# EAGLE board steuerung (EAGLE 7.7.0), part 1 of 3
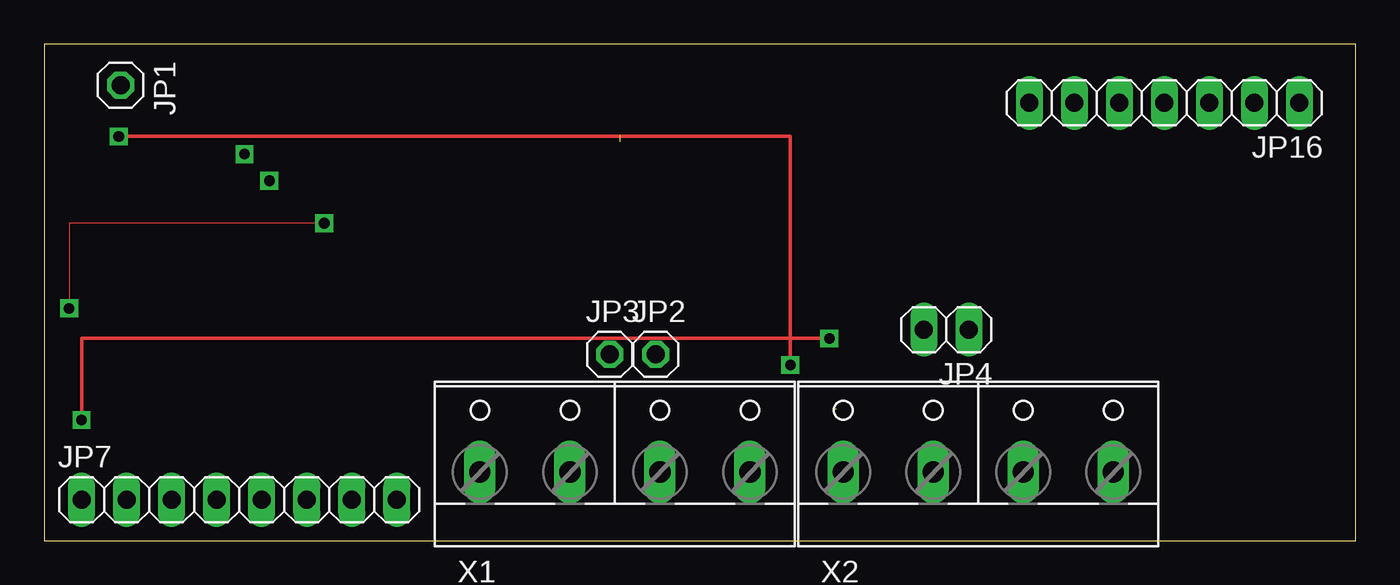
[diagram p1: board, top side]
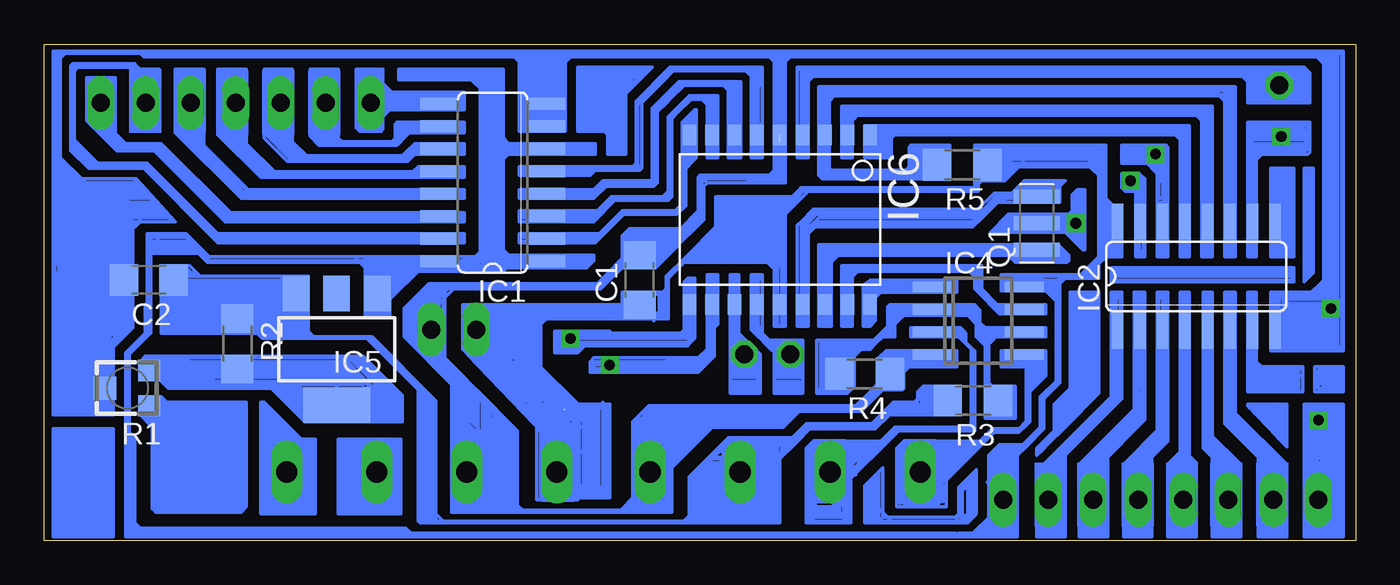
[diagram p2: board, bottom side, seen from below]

Size 74 x 28 mm. Coordinates in mm from the lower left corner, seen from the top.
Outline: 0,0 74,0 74,28 0,28 0,0
Copper layers (1*16): Top 0.035mm / dielectric 1.5mm / Bottom 0.035mm
Design rules "default": minimum track width 10mil, minimum drill 24mil, track to track 8mil, track to pad 8mil, pad to pad 8mil, via to via 8mil, smd to smd 8mil, copper to edge 40mil, drill to drill 8mil, minimum pad ring 10mil, minimum via ring 8mil, stop-mask expansion 4mil, vias tented up to drill 0mil, thermal gap 10mil

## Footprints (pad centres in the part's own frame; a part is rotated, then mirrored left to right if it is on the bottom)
C1206 = smd 1.6 x 1.8: 1 -1.4,0; 2 1.4,0
SO16 = smd 0.66 x 2.032: 1 -4.445,-3.073; 2 -3.175,-3.073; 3 -1.905,-3.073; 4 -0.635,-3.073; 5 0.635,-3.073; 6 1.905,-3.073; 7 3.175,-3.073; 8 4.445,-3.073; 9 4.445,3.073; 10 3.175,3.073; 11 1.905,3.073; 12 0.635,3.073; 13 -0.635,3.073; 14 -1.905,3.073; 15 -3.175,3.073; 16 -4.445,3.073
SO08 = smd 0.6 x 2.2: 1 -1.905,-2.6; 2 -0.635,-2.6; 3 0.635,-2.6; 4 1.905,-2.6; 5 1.905,2.6; 6 0.635,2.6; 7 -0.635,2.6; 8 -1.905,2.6
SOT223 = smd 1.5 x 2: 1 -2.3,-3.15; 2 0,-3.15; 3 2.3,-3.15 | smd 3.8 x 2: 4 0,3.15
SO-18W = smd 0.762 x 1.143: 1 -5.08,-4.788; 2 -3.81,-4.788; 3 -2.54,-4.788; 4 -1.27,-4.788; 5 0,-4.788; 6 1.27,-4.788; 7 2.54,-4.788; 8 3.81,-4.788; 9 5.08,-4.788; 10 5.08,4.788; 11 3.81,4.788; 12 2.54,4.788; 13 1.27,4.788; 14 0,4.788; 15 -1.27,4.788; 16 -2.54,4.788; 17 -3.81,4.788; 18 -5.08,4.788
1X01 = drill 1.016 octagon: 1 0,0
1X02 = drill 1.016 long: 1 -1.27,0; 2 1.27,0
1X08 = drill 1.016 long: 1 -8.89,0; 2 -6.35,0; 3 -3.81,0; 4 -1.27,0; 5 1.27,0; 6 3.81,0; 7 6.35,0; 8 8.89,0
1X07 = drill 1.016 long: 1 -7.62,0; 2 -5.08,0; 3 -2.54,0; 4 0,0; 5 2.54,0; 6 5.08,0; 7 7.62,0
CSTCR6M = smd 0.8 x 2.6: 1 -1.5,0; 2 0,0; 3 1.5,0
RTRIM3103 = smd 1.2 x 1.25: 1 -1,-1.225; 3 1,-1.225 | smd 1.3 x 1.3: 2 0,1.3
R1206 = smd 1.6 x 1.803: 1 -1.422,0; 2 1.422,0
W237-4P = drill 1.194 long: 1 -7.62,-0.635; 2 -2.54,-0.635; 3 2.54,-0.635; 4 7.62,-0.635

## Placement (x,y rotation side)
C1  100n  [C1206]  40.4,14.7 90 bottom
C2  100n  [C1206]  68.1,14.7 180 bottom
IC1  4543D  [SO16]  48.7,20.2 90 bottom
IC2  4028D  [SO16]  9,14.9 0 bottom
IC4  LM358D  [SO08]  21.3,12.4 270 bottom
IC5  LM317  [SOT223]  57.5,10.8 180 bottom
IC6  PIC18F1220SO  [SO-18W]  32.5,18.1 180 bottom
JP1  [1X01]  4.3,25.7 270 top
JP2  [1X01]  34.5,10.5 0 top
JP3  [1X01]  31.9,10.5 0 top
JP4  [1X02]  50.9,11.9 180 top
JP7  [1X08]  11,2.3 0 top
JP16  [1X07]  63.2,24.7 180 top
Q1  CSTCR6M00G53Z  [CSTCR6M]  18,17.9 90 bottom
R1  5k  [RTRIM3103]  69.3,8.6 90 bottom
R2  220  [R1206]  63.1,11.1 270 bottom
R3  10k  [R1206]  21.6,7.9 180 bottom
R4  10k  [R1206]  27.7,9.4 180 bottom
R5  1k  [R1206]  22.2,21.2 180 bottom
X1  [W237-4P]  32.2,4.5 0 top
X2  [W237-4P]  52.7,4.5 0 top

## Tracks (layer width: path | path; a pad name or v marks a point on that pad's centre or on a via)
N$1
  Bottom 0.2: 70.5,25.8 70.1,25.8 | 70.1,25.8 70.1,26.1 | 71.5,26.1 71.6,26.1 71.6,23.7 69.9,22 69.7,22 69.6,22.1 | 70.8,23.2 69.6,22 | IC1.14 50.41,18.3 50.3,18.4 | 50.3,18.4 50.3,18.5 63.6,18.5 67.6,22.4 | 67.6,22.4 69.4,22.4 | 69.4,22.4 70.1,23.1 70.1,23.3 | 70.1,23.8 70.1,23.98 | 70.1,23.98 JP16.1 | 50.3,18.4 50.3,18 63.8,18 67.8,22 69.5,22 | 69.5,22 69.6,22.1 | 69.6,22.1 70.4,22.9 | 70.4,22.9 70.7,23.2 | 70.7,23.2 70.6,23.2 | 70.4,23.2 70.3,23.1 | 70.3,23.1 70.3,23 69.5,22.2 69.4,22.2 | 69.4,22.2 67.5,22.2 63.8,18.5 63.8,18.4 | 63.8,18.4 64,18.4 | 64,18.4 67.7,22.1 | 69.4,22.2 70,22.8 | 70.1,22.9 70.3,23.1 | 69.6,22 69.5,22 | 63.8,18.4 63.4,18.4 | 63.4,18.4 50.5,18.4 50.5,18.3 50.4,18.2 50.4,18.4 50.5,18.5 50.5,18.2 50.4,18.1 63.7,18.1 63.8,18.2 | 64,18.4 63.8,18.2 | 63.8,18.2 52.5,18.2 52.4,18.3 | 69.4,22.2 69.6,22 | 69.6,22 69.8,22 70.9,23.1 | 69.6,22.1 69.5,22.1 69.3,22.3 69.4,22.4 | 70.1,24.5 70.1,25.8 | 71.3,26.1 71.5,26.1 | 71.5,26.1 71.5,24 70.7,23.2 | 70.4,22.9 70.1,22.9 | 70.1,22.9 70,22.8 | 70,22.8 70,26.1 70.1,26.1 | 70.1,26.1 70.2,26.1 | 70.5,26.1 71.3,26.1 | 71.4,26 71.3,26.1 | 71.3,26.1 71.3,24.5 | 71.3,24.3 71.3,24.1 71.4,24 | 71.4,24 71.5,23.9 71.5,23.8 70.5,22.8 70.5,23 70.4,23.1 70.3,23.1 | 70.3,23.1 70.2,23.2 | 70.2,24.3 70.2,24.5 | 70.2,24.5 70.3,24.6 70.5,24.6 | 71.1,24.6 71.2,24.6 71.3,24.5 | 71.3,24.5 71.3,24.3 | 71.3,24.3 71,24 | 70.2,23.2 70.2,23.4 | 70.2,23.4 70.2,23.6 | 70.2,23.6 70.2,24.3 | 70.2,24.3 70.5,24.6 | 70.5,24.6 71.1,24.6 | 71.1,24.6 71.2,24.7 71.1,24.7 70.3,23.9 70.3,23.7 70.2,23.6 | 70.2,23.6 70.3,23.6 | 70.3,23.6 71.2,24.5 71.2,24.1 70.9,24.1 | 70.9,24.1 70.3,23.5 | 70.2,23.4 70.1,23.3 | 70.1,23.3 70.3,23.3 | 70.3,23.3 70.5,23.3 71.2,24 71.2,26.1
  Bottom 0.2: 70.5,26.1 70.3,26.1 | 70.3,26.1 70.3,23.5 | 70.3,23.5 70.2,23.4 | 70.2,24.5 70.2,26.1 | 70.2,26.1 70.3,26.1 | 70.3,26.1 70.4,26 | 70.4,26 70.6,26 70.6,23.4 70.4,23.2 | 70.4,23.2 70.6,23.2 | 70.6,23.2 71.4,24 | 71.4,24 71.4,25.9 71.2,26.1 | 71.2,26.1 71.1,26.1 | 71.1,26.1 70.5,26.1 | 70.5,26.1 70.4,26 | 70.4,26 70.4,23.4 | 70.4,23.4 70.3,23.3 | 70.3,23.3 70.2,23.2 | 70.2,23.2 70.5,23.2 70.7,23.4 70.7,25.8 70.9,26 71,26 | 71,26 71.1,26.1 | 71.1,26.1 71.1,24.2 70.8,23.9 70.8,25.5 70.9,25.6 | 70.9,25.6 70.9,24.1 | 70.9,25.6 70.9,25.9 71,26 | 71,26 71,24 | 71,24 70.4,23.4 | 70.3,23.3 70.3,23.6 | 70.3,23.6 70.1,23.8 | 70.1,23.8 70.1,23.3 | 70.1,23.98 70.1,24.5 | 70.1,24.5 70.5,24.9 | 63.4,18.4 67.4,22.4 67.6,22.4
N$2
  Bottom 0.2: 63.5,23 63.4,23 | 63.4,23 63.2,23 | 63.2,23 62.7,22.5 62.7,22.7 62.8,22.8 63.2,22.8 63.4,23 | 63.2,23 62.9,23 62.7,22.8 63.1,22.8 63.2,22.7 63.1,22.7 61.1,20.7 53.2,20.7 | 53.2,20.7 52.9,20.7 52.9,20.9 53,20.9 | 53,20.9 53.2,20.7 | 53,20.9 52.9,21 50.5,21 50.4,20.9 50.4,20.8 50.5,20.7 51.9,20.7 52,20.8 50.6,20.8 50.5,20.9 50.5,20.8 50.4,20.7 50.4,20.6
N$3
  Bottom 0.2: IC6.8 36.31,22.69 36.6,22.4 | 36.6,22.4 36.6,21.6 36,21.6 36,24.1 | 36,24.1 36.3,24.1 | 36.4,24.1 36.6,24.1 | 41.7,19.4 42,19.4 42.8,18.6 47.2,18.6 47.2,18 43,18 41.8,19.2 38.8,19.2 38.6,19.4 38.6,23.8 38.3,24.1 | 39.1,19.4 38.9,19.4 | 38.9,19.4 38.8,19.5 38.8,19.7 | 38.8,19.7 38.8,23.9 38.4,24.3 | 38.4,24.3 38.3,24.3 38.6,24 38.6,23.7 38.7,23.6 38.7,19.5 38.8,19.4 38.9,19.4 | 36.6,24.1 36.6,23.9 | 36.6,22.4 36.6,23.9 | 36.6,23.9 36.5,24 | 36.5,23.8 36.5,21.7 36.4,21.7 36.3,21.8 36.3,23.7 | 36.3,24 36.4,24.1 | 36.4,24.1 36.3,24.1 | 36.3,24.1 36.2,24 36.2,23.8 | 36.2,23.8 36.2,21.7 36.1,21.7 36.1,24 36,24.1 | 36,24.1 36,24.3 | 39.1,19.4 41.7,19.4 | 41.7,19.4 41.9,19.2 42,19.2 43.1,18.1 45.43,18.1 IC1.3 | 38.8,19.7 39.1,19.4 | 36.3,23.7 36.5,23.7 | 36.3,23.7 36.3,24 | 36.3,24 36,24.3 | 36,24.3 36,25.1 37.6,25.1 38.4,24.3 | 36.6,24.1 36.6,24.9 37.5,24.9 38.3,24.1 | 38.3,24.1 38.3,24.2 37.6,24.9 37.6,25 37,25 | 37,25 36.2,25 36.1,24.9 36.1,23.9 36.2,23.8 | 36.2,23.8 36.5,23.8 | 36.5,23.8 36.5,24.9 36.4,24.9 36.3,24.8 | 36.3,24.8 36.3,24.2 36.3,24.1 | 36.3,24.8 36.3,24.9 | 36.3,24.1 36.4,24 36.4,24.4 37,25
N$4
  Bottom 0.2: 7,10.8 6.9,10.9 6.8,10.9 6.8,14 7.4,14 7.4,6.8 | 7.4,6.8 7.4,6.7 | 7.4,6.7 5.5,4.8 5.4,4.7 | 5.4,4.7 5,4.3 | 7.3,7.5 7.3,6.9 7.4,6.8 | 7.4,6.7 7.4,6.6 5.1,4.3 | 5.4,4.1 5.4,4.7
N$5
  Bottom 0.2: IC2.13 9.73,23.23 11.2,23.3 27.42,23.2 IC6.1
N$6
  Bottom 0.2: 14.6,15.5 14,16.1 14.1,16.1 14.5,15.7 | IC6.14 32.6,13.31 32.6,18.9 32,18.9 33.6,18 32.47,19.17 | 32.47,19.17 32.5,19.2 | 14.3,18.8 14.4,18.7 14.2,18.5 | 16.8,13.6 17.3,14.1 16.8,14.6 | 16.8,13.6 16.8,8.9 17.7,8 17.7,6.3 18.5,5.5 18.5,5.4 18.9,5 19.1,5 19.9,4.2 JP7.8 | 14.2,18.5 14.2,18.2 14.1,18.2 14.1,18.4 14.2,18.4 14.2,17.2 14.4,17.2 14.4,17 14.3,17 14.3,16.9 | 14.2,18.5 14.2,21.7 14.6,22.1 20,22.1 20.4,21.7 20.4,21.4 21.4,20.4 | 21.4,20.4 21.5,20.3 21.5,19.9 | 21.5,19.9 31.3,19.9 | 31.3,19.9 31.6,19.4 31.8,19.4 | 31.8,19.4 32.24,19.4 32.47,19.17 | 21.4,20.4 21.4,19.9 21.5,19.8 21.5,19.9 | 31.3,19.9 31.8,19.4 | 14.2,16.8 13.2,16.8 13.2,16.1 | 13.2,16.1 13.2,16 14.4,16 | 14.4,16 14.5,16 | 14.5,16 14.7,15.8 14.7,14.8 | 14.7,14.8 16.4,14.8 | 16.4,14.8 16.5,14.8 | 16.5,14.8 16.6,14.8 16.8,14.6 | 16.8,13.6 16.8,14.5 16.5,14.8 | 13.2,16.1 14.3,16.2 | 14.3,16.2 14.4,16.3 13.5,16.3 13.4,16.2 14.3,16.2 | 14.3,16.2 14.4,16.2 14.2,16.5 14.5,16.4 | 13.9,16.4 14.5,16.4 | 14.5,16.4 14.3,16.6 14.5,16.5 | 14.5,16.5 14.3,16.7 | 14.3,16.7 14.1,16.7 | 14.1,16.7 14,16.6 14.2,16.6 14.3,16.5 14.4,16.5 14.3,16.7 | 14.3,16.7 14.3,16.9 | 14.3,16.9 14.2,16.8 | 14.2,16.8 14.1,16.7 | 16.8,14.6 16.6,14.6 16.4,14.8 | 14.7,14.8 14.5,14.8 14.5,15.7 | 14.5,15.7 14.5,15.9 14.4,16 | 14.3,16.2 14.5,16 | 14.5,16 14.5,16.4 | 14.5,16.4 14.5,16.5 | 14.5,16.5 14.5,16.6
N$7
  Bottom 0.2: IC2.5 8.37,5.5 7.87,5 7.87,2.98 JP7.3
N$8
  Bottom 0.2: 37.9,19 38.4,18.5
N$9  (via drill 0.6)  (1 unrouted)
  Top 0.05: v15.8,17.9 1.4,17.9 v1.4,13.1
  Bottom 0.05: v1.4,13.1 1.4,12.3
  Bottom 0.2: 15.5,18.3 15.4,18.3 | 15.4,18.3 15.3,18.4 | 15.3,18.4 15.3,16.4 15.4,16.4 16,17 | 16,17 16,17.2 | 16,17.5 16,17.6 | 16,17.6 16,17.7 | 16,17.7 v15.8,17.9 | v15.8,17.9 15.4,18.3 | 15.3,18.4 15.3,19.8 15.7,19.8 16,19.5 16,18.6 | 16,18.6 16.3,18.3 19.6,18.3 | 19.6,18.3 19.6,18.1 | 19.6,18.1 19.6,17.5 | 19.6,17.5 16.5,17.5 16,17 | 16,18.6 16,18.2 | 16,18.2 16,17.7 | 16,17.2 15.6,16.8 | 15.6,16.8 15.4,16.6 15.4,19.7 15.7,19.7 15.7,19.6 15.9,19.4 15.8,19.4 15.6,19.6 15.6,17.9 | 15.6,17.9 15.6,16.9 | 15.6,16.8 15.6,16.9 | 15.6,16.9 15.8,17.1 15.8,17.6 | 15.8,17.6 v15.8,17.9 | v15.8,17.9 15.8,19.3 15.7,19.4 15.7,18.5 15.9,18.3 | 15.9,18.3 16,18.2 | 16,18.2 19.3,18.2 19.4,18.1 19.4,17.6 19,17.6 | 16.2,17.6 16.1,17.6 | 16.1,17.6 16,17.5 | 16,17.5 16,17.2 | 50.9,9.7 52,10.8 52,13.6 51.4,14.2 | 51,9.5 51,9.6 51.4,10 | 51.4,10 52.2,10.8 52.2,10.9 | 52.2,10.9 52.2,11.5 | 52.2,11.5 52.2,11.8 | 52.2,12.9 52.2,14.1 52.1,14.2 51.7,14.2 52.1,13.8 52.1,14 52,14.1 52.3,14.4 | 52.2,10.9 51.5,10.2 | 71.4,14 70.7,14 69.2,15.5 69.2,17.4 | 69.2,17.6 69.2,18.2 | 69.2,18.2 69.2,18.5 | 69.2,18.5 69.2,19.1 67.9,19.1 67,18.2 68.6,18.2 | 68.6,18.2 69.2,18.2 | 69.2,18.2 69.1,18.1 69.1,18.5 | 69.1,18.6 69.1,18.9 67.8,18.9 67.3,18.4 69,18.4 69.1,18.5 | 69.1,18.5 69.1,18.6 | 69.1,18.6 69,18.7 67.8,18.7 67.6,18.5 69.2,18.5 | 68.6,18.2 68.6,18 69.2,17.4 | 70.4,8.1 70.8,7.7 | 71.1,7.4 71.2,7.3 72.2,7.3 72.8,7.9 70.4,7.9 71.1,7.2 | 66.9,18.1 66.9,18.2 68.3,19.6 | 68.4,19.7 68.9,20.2 71.9,20.2 72.9,21.2 72.9,20.2 73.1,20.1 | 69,15.3 69,17.5 | 70.6,8.7 70.6,9.4 70.4,9.4 | 70.4,9.4 70.1,9.1 | 70.1,9.1 70.1,8.1 | 70.1,8.1 70.8,7.4 | 70.8,7.4 71,7.2 | 70.4,9.4 71.1,10.1 71.1,7.4 | 71.1,7.2 71.1,7.1
  Bottom 0.2: 71.1,7.1 72.1,7.1 | 72.1,7.1 72.2,7.1 | 72.2,7.1 72.4,7.3 | 72.4,7.3 72.6,7.5 | 72.6,7.5 73.1,8 | 40.1,5.6 40.8,5.6 | 40.8,5.6 40.8,2.4 41.4,1.8 41.3,1.8 40.8,2.3 40.8,2.1 41.1,1.8 38.9,1.8 38.8,1.7 38.8,3.2 40.6,5 | 40.8,5.6 40.8,6.2 36.9,6.2 | 53.6,11.8 50.9,9.1 50.9,6.2 | 49.1,1.8 49.1,6.2 | 49.1,6.2 50,6.2 | 50,6.2 50.7,6.2 | 50.9,6.2 51,6.2 | 51,6.2 51,1.6 50.9,1.6 | 41.2,15.6 41.4,15.6 42.5,14.5 42.6,14.5 | 42.6,14.5 42.8,14.5 | 42.8,14.5 52,14.5 | 52,14.5 53.5,13 | 40.9,16.4 42.8,14.5 | 39,2.4 39,1.6 | 26.4,8.7 26.5,8.7 27.9,7.3 28,7.3 | 38.6,16.4 38.5,16.4 36.8,18.1 36.8,18.2 | 46.3,27 46.4,26.9 46.4,27 46.5,27.1 46.5,27.2 46.3,27.2 | 45.5,24.5 45.8,24.9 | 45.8,24.9 46.1,25.3 | 46.1,25.3 46.2,27.2 | 32.5,22.5 32.3,22.5 32.2,22.4 32.2,21.7 | 32.3,21.7 32.8,21.7 | 47.3,27.3 68.4,27.3 68.6,27.5 | 47.1,27.3 46.9,27.3 | 46.8,27.3 46.6,27.3 | 46.6,27.3 46.5,27.3 | 44.2,27.3 33.1,27.3 | 33.1,27.3 32.8,27.3 | 32.2,27.3 32,27.3 | 32,27.3 31.9,27.3 | 31.9,27.3 1.8,27.3 | 1.7,27.3 1.8,27.3 | 1.8,27.3 1.8,14.7 | 1.8,14.5 1.8,14 | IC2.8 4.55,13.35 3.9,14 | 3.9,14 1.8,14 | 1.8,14 1.4,14 | 1.4,14 1.6,27.5 | 1.6,27.5 68.1,27.5 | 4.1,13.8 4.2,13.8 | 4.2,13.8 4.5,13.8 | 4.5,13.8 4.6,13.8 4.7,13.9 4.7,10.9 | 4.7,10.9 4.8,10.9 | 4.8,10.9 4.8,14 3.9,14 | 3.9,14 3.9,13.4 | 3.9,13.2 3.9,13 | 3.9,11.8 3.9,11.6 | 3.9,11.6 3.9,10.7 | 4.8,10.9 4.8,10.7 3.9,10.7 | 4.7,10.9 4.2,10.9 | 4.2,10.9 4.1,10.9 | 4.1,10.9 4.1,13.9 | 4.2,13.8 4.3,13.7 4.3,12.5 | 4.5,13.8 4.4,13.7 4.4,12.4 | 3.9,10.7 1.4,10.7 | 1.6,27.5 1.4,27.5 | 1.4,27.5 1.4,14 | 1.4,14 1.4,13.2 | 1.4,13.2 v1.4,13.1 1.4,13 | 1.4,13 1.4,12.8 | 1.4,12.8 1.4,12.7 | 1.4,12.1 1.4,12 | 1.4,12 1.4,11.7 | 1.4,11.7 1.4,11.1 | 1.4,10.8 1.4,10.7 | 32.5,27 32.5,23.3 32.6,23.4 32.6,27 32.7,27.1
  Bottom 0.2: 32.5,27 32.8,27.3 | 1.4,13 1.7,13 | 3.8,13 3.9,13 | 3.9,13 3.9,12.1 | 3.9,12.1 3.9,11.8 | 3.9,11.8 3.6,11.8 | 3.6,11.8 1.6,11.8 | 1.6,11.8 1.5,11.8 | 1.4,13.2 1.8,13.2 | 1.8,13.2 1.9,13.2 | 1.9,13.2 3.4,13.2 | 3.4,13.2 3.6,13.2 | 3.6,13.2 3.9,13.2 | 3.9,13.2 3.9,13.4 | 3.9,13.4 1.5,13.4 1.5,13.6 3.9,13.6 4,13.5 4,13.8 2.7,13.8 | 2.7,13.8 1.5,13.8 | 1.4,11.7 3.4,11.7 | 3.6,11.7 3.8,11.7 3.9,11.6 | 3.9,11.6 3.8,11.5 1.5,11.5 1.5,11.3 4.1,11.3 | 4.1,10.8 4.2,10.9 | 4.2,10.9 4.2,11.3 | 4.2,11.3 4.2,13 4,12.8 4,12.7 | 4,12.7 4,12.6 | 4,12.6 4,12.1 | 4,12.1 4,11.6 | 4,11.6 4,11.2 | 4,11.2 4,10.8 | 4.2,11.3 4.1,11.3 | 4.1,11.3 4,11.2 | 4,11.2 1.5,11.2 1.4,11.1 | 1.4,11.1 1.5,11 4.1,11 4.2,10.9 | 4.1,10.9 1.6,10.9 | 1.6,10.9 1.5,10.9 | 1.8,13.2 1.4,12.8 | 1.4,12 1.6,11.8 | 4,11.6 3.5,11.6 3.4,11.7 | 3.4,11.7 3.6,11.7 | 3.6,11.7 3.8,11.9 | 3.8,11.9 4,12.1 | 3.6,13.2 3.6,13.1 4,12.7 | 3.4,13.2 4,12.6 | 3.9,12.1 3.6,11.8 | 2,11.6 1.9,11.6 1.6,11.9 | 1.6,11.9 1.4,12.1 | 1.4,12.1 1.4,12.3 1.4,12.7 | 1.4,12.7 1.6,12.9 | 1.7,13 1.9,13.2 | 1.6,13.1 1.6,12.9 | 1.6,12.2 1.6,11.9 | 1.6,11.9 3.8,11.9 | 3.8,11.9 3.8,12.1 | 3.8,12.1 3.8,13 | 3.8,13 1.8,13 | 1.8,13 1.7,13 | 1.7,13 1.6,12.9 | 1.6,12.9 1.6,12.2 | 1.6,12.2 1.7,12.1 3.7,12.1 | 3.8,12.1 3.7,12.1 | 3.7,12.1 3.6,12.2 | 3.6,12.8 3.6,13 3.7,13.1 1.9,13.1 1.8,13 | 1.8,13 1.8,12.7 | 1.8,12.7 1.8,12.3 1.7,12.2 3.6,12.2 | 3.6,12.2 3.6,12.5 | 3.6,12.5 3.6,12.8 | 3.6,12.8 3.5,12.9 1.7,12.9 | 3.6,12.8 3.7,12.7 3.4,12.7 | 1.8,12.7 3.4,12.7 | 3.4,12.7 3.6,12.5 | 32.8,21.7 32.8,21.8 | 32.8,21.8 32.8,27.3 | 32.8,27.3 32.4,27.3 | 32.4,27.3 32.2,27.3 | 32.2,27.3 32.2,21.8 32.3,21.7 | 32.3,21.7 32.3,26.9 | 32.3,27 32.3,27.2 32.4,27.3 | 32.4,27.3 32.5,27.2 32.5,27 | IC1.8 46.45,24.64 46.7,24.9 46.7,26
  Bottom 0.2: 46.7,26 46.7,26.3 | 46.7,26.3 46.7,26.5 | 46.7,26.5 46.7,27.2 46.8,27.3 | 47.2,24.4 47.2,27.2 47.3,27.3 | 47.3,27.3 47.1,27.3 | 47.1,27.3 47,27.2 47,24.6 47.1,24.5 | 47.1,24.5 46.9,24.5 | 46.9,24.5 46.8,24.6 46.8,25.9 | 46.8,26.2 46.8,26.4 | 46.8,26.4 46.8,27.2 46.9,27.3 | 46.9,27.3 46.8,27.3 | 44.2,27.3 46,27.2 | 44.2,27.3 44.3,27.3 | 46.2,27.3 46.4,27.3 | 46.4,27.3 46.5,27.3 | 46.5,27.3 46.6,27.2 | 46.5,25 46.6,25.1 46.6,25.9 | 46.4,27.3 46,27.2 | 46,27.2 46.2,27.2 | 46.2,27.2 46.3,27.2 | 46.5,26.9 46.5,26.8 | 46.5,25.3 46.5,25.2 46.4,25.1 | 46.5,26.8 46,25.7 46.6,25.7 46.8,25.9 | 46.1,25.3 46.5,25.3 | 46.5,25.3 46.5,26.4 | 46.5,26.4 46.5,26.8 | 46.6,25.9 46.6,27.3 | 45.9,26.4 45.9,26.2 | 46.8,25.9 46.8,26.2 | 46.8,26.2 46.7,26.3 | 45.9,26.4 46.5,26.4 | 46.7,26.3 46.8,26.4 | 46.8,26.4 46.5,26.4 | 46.7,26 46.6,25.9 | 46.6,25.9 45.9,26.4 | 32.8,21.7 32.8,21.6 | 32.8,21.6 32.5,21.6 | 32.5,21.6 32.2,21.6 | 32.2,21.6 32.3,21.7 | 32.3,21.7 32.2,21.7 | 32.2,21.7 32.2,21.6 | 32.3,26.9 32.3,27 | 32.3,27 32,27.3 | 31.9,27.3 32.3,26.9 | 32.4,26.7 32.5,26.7 33.1,27.3 | 68.2,27.4 68.1,27.5 | 68.1,27.5 68.2,27.5 68.3,27.4 | 68.3,27.4 68.6,27.6 | 72.5,27.6 73.1,27.5 | 68.7,27.6 68.6,27.5 | 68.6,27.5 68.5,27.5 | 68.6,27.6 68.5,27.5 | 68.4,27.4 68.5,27.5 | 68.5,27.5 68.5,27.6 68.3,27.4 | 68.6,27.6 68.7,27.6 | 68.6,27.5 68.6,27.6 | 68.7,27.6 72.5,27.6 | 72.5,27.6 72.6,27.6 | 72.6,27.6 73.1,27.5 | 73.1,27.5 73.1,27.2 | 68.6,27.5 73.1,27.5 | 73.1,27.2 73.1,24.7 | 73.2,27.1 73.2,24.8 73.1,24.7 | 73.2,27.1 73.1,27.2 | 73.1,27.2 72.7,27.6 | 72.7,27.6 72.6,27.6 | 68.6,27.6 1.4,27.6 | 1.4,27.6 1.4,27.5 | 72.7,27.6 72.8,27.6 | 72.8,27.6 73.2,27.2 73.2,27.1 | IC4.4 25.18,10.49 R4.1 26.28,9.22 28.2,7.3 | 39.1,4.58 X1.4 39.9,3.94 39.9,4.6
  Bottom 0.2: 33,20.6 32.5,20.6 32.5,21.6 | 73.1,21.6 73.1,20.1 | 73.1,20.1 73.1,14 | 73.1,14 73.1,13.8 | 73.1,13.8 73.1,13.7 | 73.1,13.7 73.1,12 | 73.1,12 72,10.9 71.85,11 R1.2 | C2.2 69.55,14.65 72.95,14.65 73,14.6 | 41.1,17.2 41.4,16.9 | 41.4,16.9 41.2,16.9 41.15,16.85 | 41.15,16.85 41.1,16.8 | 40.8,16.5 C1.2 | 41.4,16.9 41.4,15.7 | 41.4,15.7 41.4,15.4 | 41.4,15.4 39.5,15.4 38.2,16.7 | 32.5,20.2 32.3,20.4 | 32.3,20.4 32.3,21.5 32.2,21.6 | 32.2,21.6 32.2,20.5 | 32.2,20.5 32.3,20.4 | 32.5,20.2 33.9,20.2 | 33.9,20.2 34.1,20.4 32.6,20.4 32.6,21.9 32.7,21.9 32.8,21.8 | 32.8,21.6 32.8,20.9 33.1,20.6 | 33.1,20.6 33,20.6 | 33,20.6 32.7,20.9 32.7,20.7 32.4,20.4 32.5,20.3 34.1,20.3 | 34.3,20.2 34.3,20.3 34.2,20.4 | 41.1,17 41,17.1 41,17 | 39.5,16.9 39.8,16.6 39.8,15.9 39.5,15.6 38.3,16.8 | 38.3,16.8 38.4,16.8 | 38.4,16.8 39.4,16.8 39.5,16.7 39.5,16.4 | 39.5,16.4 39.5,15.8 | 39.5,15.7 39.5,15.8 | 39.5,15.8 38.6,16.7 38.8,16.7 | 39.2,16.7 39.3,16.6 39.3,16.2 | 39.3,16.2 39.4,16.1 | 39.3,16.2 38.8,16.7 | 38.8,16.7 39.2,16.7 | 39.2,16.7 39.3,16.7 | 39.4,16.7 39.3,16.7 | 39.3,16.7 39.1,16.5 39.4,16.5 39.5,16.4 | 41.1,17.2 41.4,17.2 | 41.4,17.2 41.4,16.9 | 33.1,20.6 37,20.6 37.1,20.5 37.1,18.6 38.1,17.6 41,17.6 41.4,17.2 | 41.1,17.2 38.1,17.2 37,18.3 | 36.9,18.4 36.9,18.5 | 36.9,18.5 36.8,18.6 | 36.9,18.5 37.1,18.3 37,18.3 | 37,18.3 36.9,18.4 | 36.9,18.4 36.8,18.5 | 36.8,18.5 36.8,20 36.6,20.2 34.1,20.2 | 34.1,20.2 33.9,20.2 | 34.1,20.2 34.1,20.3 | 34.1,20.3 34.2,20.4 | 34.2,20.4 36.9,20.4 37,20.3 37,18.6 37.1,18.5 37.1,20 36.8,20.3 37,20.5 36.9,20.5 36.7,20.3 36.9,20.3 36.9,18.6 38,17.5 40.9,17.5 41.1,17.3 38.1,17.3 | 36.8,18.2 36.8,18.4 | 36.8,18.5 36.8,18.4 | 36.8,18.4 38.2,17
  Bottom 0.2: 38.4,16.8 38.2,17 | 38.2,17 41,17 | 41,17 41.1,17.1 41.1,16.8 | 41.1,16.8 40.8,16.5 | 40.8,16.5 39.5,16.5 39.2,16.2 | 41,17 41.15,16.85 | 36.8,18.2 36.9,18.2 38.3,16.8 | 41.4,15.4 42.4,14.4 52.3,14.4 | 28.2,7.3 31.4,7.3 32.3,6.4 36.3,6.4 37.9,4.8 39.7,4.8 39.9,4.6 | 23.2,10.6 22.6,10.6 | 22.6,10.6 22.5,10.7 | 22.5,10.7 24.9,10.7 | 24.9,10.7 25.1,10.7 | 25.1,10.7 25.1,10 | 25.1,10 23.2,10 22.6,10.6 | 22.5,10.7 22.5,9.8 25.1,9.8 25.1,10 | 25.1,10 25,10.1 22.7,10.1 | 24.7,10.6 24.8,10.6 24.9,10.7 | 25.1,10.7 26.5,10.7 26.9,10.3 26.9,8.9 | 26.9,8.9 26.9,8.5 26.8,8.5 | 26.8,8.5 25.6,8.5 25.5,8.6 25.5,9.5 25.2,9.8 25.2,10.5 26.4,10.5 26.8,10.1 26.8,10.3 26.5,10.6 25.7,10.6 25.4,10.3 25.4,10.1 | 25.4,9.7 25.4,10.1 | 25.4,10.1 25.7,10.4 26.2,10.4 26.3,10.3 | 26.3,10.3 26.7,10.3 | 26.3,10.3 25.9,10.3 25.9,9.9 26.8,9 26.8,8.9 28.3,7.4 31.5,7.4 32.3,6.6 36.1,6.6 | 36.1,6.6 36.3,6.6 36.5,6.4 | 36.5,6.4 38,4.9 39.2,4.9 39.2,5 39.1,5.1 | 39.1,5.1 38,5.1 37,6.1 | 37,6.1 36.9,6.2 | 36.4,6.7 36.2,6.7 | 36.2,6.7 32.4,6.7 31.6,7.5 28.3,7.5 28.2,7.6 | 27.6,8.2 26.9,8.9 | 28.2,7.3 28,7.3 | 28,7.3 26.8,8.5 | 39.9,4.6 39.7,4.6 39.1,5.2 39.1,5.1 | 39.1,5.1 39.1,4.1 40.3,2.9 40.3,1.7 40.4,1.6 | 40.4,1.6 40.6,1.6 | 40.6,1.6 40.9,1.6 | 40.9,1.6 48.5,1.6 | 48.5,1.6 50.1,1.6 | 50.1,1.6 50.2,1.7 50.2,3.83 X2.2 50.16,8.56 53.6,12 53.6,13.1 | 52.3,14.4 52.4,14.4 | 52.4,14.4 53.6,13.2 | 53.6,13.2 53.6,13.1 | 39,1.6 40.4,1.6 | 40.6,1.6 40.6,2.4 40.3,2.4 | 40.3,2.4 39.4,2.4 39.1,2.1 39.1,1.7 40,1.7 | 40,1.7 40.4,1.7 | 40.4,1.7 40.5,1.8 40.5,2 | 40.5,2 40.4,2.1 40.1,2.1 | 40.1,2.1 39.3,2.1 39.2,2 39.2,1.9 40.4,1.9 | 40.1,2.1 40.1,1.8 40,1.7 | 40.5,2.2 40.5,2 | 40.5,2 40.8,1.7
  Bottom 0.2: 40.8,1.7 40.9,1.6 | 40.4,1.7 40.8,1.7 | 40.8,1.7 41,1.7 | 40.3,2.4 41,1.7 | 41,1.7 47,1.7 | 48.7,1.7 48.9,1.7 49.4,2.2 50.1,2.2 50.1,1.6 | 50.1,1.6 50.9,1.6 | 50.9,1.6 50.9,2.1 | 50.9,2.2 50.9,2.1 | 50.9,2.1 50.8,2 49.4,2 49.1,1.7 50.7,1.7 50.8,1.8 49.4,1.8 | 52,14.5 52.3,14.5 52.4,14.4 | 48.5,1.6 49.4,2.5 | 51,6.2 51,8.8 53.7,11.5 53.7,13.1 53.6,13.2 | 49.2,6.1 50.6,6.1 | 50.6,6.1 50.8,6.1 50.9,6 50.7,6 | 50.7,6 49.3,6 | 49.3,6 49.2,5.9 49.5,5.9 49.6,5.8 | 49.6,5.8 50.9,5.8 | 49.6,5.8 49.4,5.8 | 49.4,5.8 49.2,5.8 | 50.9,6.2 50.7,6.2 | 50.7,6.2 50.6,6.1 | 50.6,6.1 50.6,8.6 53.6,11.6 53.4,11.6 50.7,8.9 50.7,6 | 50.5,5 50.5,6.9 | 50.5,6.9 50.5,7 | 50.5,7 50.5,9.2 50.9,9.6 50.9,9.5 50.4,9 50.4,8.9 | 42.2,14.7 42.2,14.6 42.6,14.2 50.9,14.2 | 51.2,14.2 51.4,14.2 | 51.4,14.2 51.5,14.2 51.9,13.8 51.9,10.8 51.5,10.4 | 51.4,10.3 50.7,9.6 | 50.7,9.6 50.2,9.1 | 50.2,9.1 50.1,9 | 50.1,9 50.1,8.6 | 50.1,6.9 50.1,4.7 50.2,4.6 | 50.4,5.5 50.4,8.9 | 50.4,8.9 50.3,9 | 50.3,9 50.2,9.1 | 50.3,9 50.3,8.9 | 50.3,8.9 50.3,6.2 | 50.3,6.2 50.3,5.6 | 50.3,6.2 49.7,5.6 | 50.6,9.1 50.5,9.1 50.3,8.9 | 50,6.2 50,6.4 50.5,6.9 | 49.4,5.8 49.4,5.9 | 49.4,5.9 50.5,7 | 39,1.6 38.6,1.6 38.6,4.5 | 38.6,4.5 38.6,5.5 38.7,5.6 38.9,5.6 38.8,5.5 38.8,4.1 | 38.8,3.9 38.8,1.8 | 37.8,5 37.8,4.9 38.8,3.9 | 38.8,3.9 38.8,4.1 | 38.8,4.1 38.2,4.7 38.5,4.7 38.5,4.6 38.6,4.5 | 36.9,6.2 36.4,6.7 | 37,6.1 40.5,6.1 40.6,6 40.6,5.8 37.5,5.8 37.3,6 40.7,6 | 36.1,6.6 36.2,6.7 | 36.4,6.7 40.5,6.7 40.6,6.6 | 40.7,6.5 40.8,6.4 | 40.8,6.4 40.8,6 40.7,5.9 | 40.7,5.9 40.7,4.8 | 40.7,5.9 40.7,6.3 | 40.7,6.3 40.7,6.5 | 40.7,6.5 40.6,6.6 | 40.6,6.6 36.7,6.6 36.5,6.4 | 36.5,6.4 40.6,6.4 40.7,6.3 | 49.4,5.7 49.4,5.8 | 49.4,5.9 49.3,6
  Bottom 0.2: 49.2,6.1 49.1,6.2 | 49.1,6.2 49.1,8 50.1,9 | 50.7,9.6 50.7,9.4 50,8.7 | 50,8.7 49.2,7.9 49.2,7.5 | 49.2,6.3 49.2,6.1 | 49.2,6.1 49.3,6 | 49.3,6 49.3,7.8 49.5,8 | 50,8.5 50.1,8.6 | 50.1,8.6 50.1,8.5 | 50.1,8.5 50.1,8.3 | 49.8,6.6 49.5,6.3 49.5,7.8 49.6,7.9 49.7,7.9 | 49.7,7.9 50,8.2 | 50,8.2 50,8 | 50,8 50,6.9 49.7,6.6 49.7,7.9 | 50,8.2 50.1,8.3 | 50.1,8.3 50.1,6.9 | 50.1,6.9 49.8,6.6 | 49.8,6.6 49.8,7.8 50,8 | 73.1,24.7 73.1,21.6 | 73.1,20.1 73,20 | 73,19.7 73,19.6 | 73,19.3 73,14.6 | 73,14.6 73,13.9 | 73,13.9 73,13.8 | 73,13.8 73.1,13.7 | 73.1,24.7 73.2,13.8 | 73.1,8 73.1,12 | 73.1,13.8 73.2,13.8 | 73.2,13.8 73.2,8.1 | 73.2,8.1 73.1,8 | 73.1,14 73,13.9 | 73,13.8 73,8.1 72.9,8 | 70.7,8.8 70.4,8.8 70.1,9.1 | 70.1,9.1 70.1,10.9 69,12 69,13.8 68.9,13.9 | 69,17.5 71.9,20.4 | 71.9,20.4 73.1,21.6 | 69,17.5 69,18 68.8,18 | 68.8,18 66.6,18 68.8,20.4 71.9,20.4 | 73.1,20.1 72,20.1 | 71.9,20.1 72,20.1 | 72,20.1 72.8,20.9 72.8,20.3 72.5,20.3 | 72.3,20.3 72.5,20.3 | 72.5,20.3 72.7,20.5 72.7,20.6 | 72.7,20.7 72.7,20.6 | 72.7,20.6 72.5,20.4 72.5,20.3 | 72.5,20.3 72.9,19.9 68.7,19.9 68.6,19.8 68.6,20 68.9,20.3 68.9,20.1 68.8,20 73,20 | 73,20 73,19.7 | 73,19.7 68.4,19.7 | 68.4,19.7 68.3,19.6 | 68.3,19.6 73,19.6 | 73,19.6 73,19.3 | 73,19.3 68.2,19.3 | 68.1,19.3 68.2,19.3 | 68.2,19.3 68.3,19.4 72.9,19.4 | 71.1,7.2 71.1,7.4 | 71.1,7.4 70.8,7.7 | 70.8,7.7 72.4,7.7 | 72.5,7.7 72.4,7.7 | 72.4,7.7 72.2,7.5 71.2,7.5 | 72.1,7.4 72.1,7.1 | 72.2,7.1 73.2,7.1 | 73.2,7.1 73.2,7.4 | 73.2,8.1 73.2,7.4 | 73.2,7.4 73.1,7.3 72.7,7.3 | 72.4,7.3 72.7,7.3 | 72.7,7.3 73.1,7.7 73.1,7.8 | 73.1,7.9 73.1,7.8 | 73.1,7.8 72.8,7.5 | 72.8,7.5 73.1,7.5 | 72.8,7.5 72.6,7.5 | 70.1,8.1 70.1,7.1 71.1,7.1 | 71.1,7.1 71,7.2 | 71,7.2 70.3,7.2 70.2,7.3 70.2,7.7 70.3,7.8 70.3,7.3 70.7,7.3 70.8,7.4
  Bottom 0.2: 70.8,7.4 70.5,7.4 70.4,7.5 70.4,7.6 70.5,7.5 | 69.2,17.4 69.2,17.6 | 69.2,17.6 68.8,18 | 47.2,24.4 44.6,24.4 | 44.6,24.4 44.6,27 44.3,27.3 | 44.3,27.3 46.2,27.3 | 46.2,27.3 46.3,27.2 | 46.3,27.2 46.3,25 46.4,24.9 45.8,24.9 | 45.8,24.9 44.9,24.9 44.8,25 44.8,27 44.6,27.2 45.7,27.2 | 45.7,27.2 46,27.2 | 46,27.2 46.1,27.1 46.1,25.1 46.2,25 46,25 | 45.1,25 45,25 44.9,25.1 44.9,27.1 45.1,27.1 | 45.8,27.1 45.9,27.1 46,27 46,25 | 46,25 45.1,25 | 45.1,25 45,25.1 45,27 45.1,27.1 | 45.1,27.1 45.8,27.1 | 45.8,27.1 45.9,27 45.9,25.4 45.7,25.2 | 45.7,25.2 45.6,25.2 | 45.6,25.2 45.3,25.2 45.2,25.1 45.2,27 45.5,27 | 45.5,27 45.8,27 45.2,26.9 45.8,24.9 | 45.8,24.9 45.4,25.3 45.4,26.9 45.6,26.9 45.6,25.2 | 41.4,15.7 42.6,14.5 | 2.7,13.8 1.8,14.7 | 1.8,14.7 1.8,14.5 | 1.8,14.5 2.4,13.9 2.2,13.9 1.7,14.4 | 1.6,10.9 1.4,10.7 | 1.4,10.7 1.3,10.7 | 1.3,10.7 1.3,27.5 | 1.3,27.5 1.3,27.6 | 1.3,27.6 1.4,27.6 | 32.2,20.5 32.2,20.2 32.5,20.2 | 27.4,8.2 27.6,8.2 | 27.6,8.2 28.2,7.6 | 28.2,7.6 39.9,7.6 40.8,6.7 40.8,6.5 | 40.8,6.4 40.8,6.5 | 40.8,6.5 40.4,6.9 40.3,6.9 | 32.4,6.9 32.1,6.9 32.1,7.1 31.8,7.4 39.8,7.4 40.3,6.9 | 40.3,6.9 32.4,6.9 | 32.4,6.9 32.1,7.2 40.1,7.2 | 40.1,7.2 40.2,7.1 32.5,7.1 32.4,7 | 39.8,7.5 40.1,7.2 | 50,8.7 50,8.5 | 50,8.5 49.5,8 | 49.5,8 49.6,8 50.1,8.5 | 50.1,8.5 49.6,8.5 47.3,6.2 47.3,2 47,1.7 | 47,1.7 48.7,1.7 | 48.7,1.7 49,2 49,6.4 | 49,7.4 49,7.7 47.4,6.1 49,6.1 49.2,6.3 | 49.2,6.3 49.2,7.5 | 49.2,7.5 48.9,7.5 47.6,6.2 47.8,6.2 | 48.7,6.2 48.8,6.2 49,6.4 | 49,6.4 49,7.4 | 49,7.4 47.8,6.2 | 47.8,6.2 48.1,6.2 | 48.6,6.2 48.7,6.2 | 48.7,6.2 48.9,6.4 48.9,7 | 48.9,7.1 48.9,7 | 48.9,7 48.8,6.9 | 48.8,6.9 48.6,6.7 | 48.3,6.4 48.1,6.2 | 48.1,6.2 48.6,6.2 | 48.6,6.2 48.8,6.4 48.8,6.7
  Bottom 0.2: 48.8,6.7 48.8,6.9 | 48.8,6.9 48.6,6.9 48,6.3 48.6,6.3 48.6,6.5 48.8,6.7 | 48.8,6.7 48.6,6.7 | 48.6,6.7 48.3,6.4 | 48.3,6.4 48.5,6.4 48.5,3 47.3,1.8 49.1,1.8 | 49.1,1.8 49.2,1.9 | 1.4,11.1 1.4,10.8 | 1.4,10.8 1.3,10.7 | 1.3,10.7 0.7,10.7 0.7,27.6 1.3,27.6 | 1.3,27.5 0.8,27.5 0.8,10.9 0.9,10.8 1.1,10.8 1.1,27.2 1.2,27.3 1.1,27.3 1,27.4 1,11 0.9,10.9 | 45.7,27.2 45.7,25.3 45.8,25.3 45.9,25.2 45.7,25.2 | 45.7,25.2 45.7,26.8 45.5,27 | 46.7,26.5 47.6,27.4 | 72.8,27.6 73.5,27.6 73.5,7.1 73.4,7.1 | 73.4,7.1 73.2,7.1 | 73.4,7.1 73.4,27.2 73.1,27.5 | 73.1,27.5 73.3,27.5 73.4,27.4 73.4,26.8 73.3,26.7 | 52.3,14.4 53.6,13.1 | JP4.1 52.17,11.53 52.2,11.5 | 51.4,14.2 51.4,10.3 | 51.4,10 51.4,10.3 | 51.4,10.3 51.5,10.4 | 51.5,10.4 51.5,13.9 | 51.5,13.9 51.7,13.7 51.7,10.7 51.6,10.6 51.6,11.2 52.2,11.8 | 52.2,11.8 52.2,12.9 | 52.2,12.9 50.9,14.2 | 50.9,14.2 51.2,14.2 | 51.2,14.2 51.5,13.9 | 51.2,14.2 51.1,14.3 | 44.6,24.4 44.6,23.1 47.2,23.1 47.2,24.4 | 47.2,24.4 47.1,24.5 | 46.9,24.5 46,24.5 | 45.5,24.5 45,24.5 44.8,24.3 44.8,24.2 | 44.8,24.1 44.8,24 | 44.8,23.8 47,23.8 47.1,23.7 47.1,23.3 46.5,23.3 46.5,23.4 46.6,23.5 | 46.6,23.5 46.8,23.7 47,23.5 46.9,23.5 | 46.9,23.5 46.8,23.4 46.7,23.4 46.6,23.5 | 46.6,23.5 46.9,23.5 | 46.9,23.5 47,23.6 47,23.9 | 47,23.9 47,24 47.1,24.1 44.8,24.1 | 44.8,24.1 44.8,24.2 | 44.8,24.2 44.9,24.3 47,24.3 47.1,24.2 47.1,24 47,23.9 | 47,23.9 44.9,23.9 44.8,24 | 44.8,24 44.8,23.8 | 44.8,23.8 44.7,23.7 | 45.5,24.5 46,24.5 | 46,24.5 46,24.2 45.63,24.2 IC1.7 | Q1.2 16.7,17.9 | 16.7,17.9 16.4,17.9 | 16,17.2 16.6,17.8 | 16.6,17.8 16.7,17.9 | 16.7,17.9 16.7,18.1 15.9,18.1 | 15.9,18.1 15.7,18.1 15.7,17.7 15.8,17.6 | 15.8,17.6 15.9,17.6
  Bottom 0.2: 15.9,17.6 16,17.6 | 16,17.6 16.1,17.6 | 16.2,17.6 16.6,17.6 | 16.6,17.6 16.8,17.8 16.6,17.8 | 16.6,17.8 16.5,17.8 | 16.5,17.8 16.4,17.9 | 16.4,17.9 16.1,17.9 | 16.1,17.9 15.9,18.1 | 15.9,18.1 15.5,18.5 15.5,18 15.6,17.9 | 15.6,17.9 15.9,17.6 | 15.9,17.6 15.9,17.7 16.1,17.9 | 16.1,17.9 v15.8,17.9 | 16.5,17.8 16.3,17.8 16.2,17.7 16.2,17.6 | 16.6,17.6 19,17.6 | 19,17.6 19.5,18.1 | 15.9,18.3 16,18.3 16.1,18.4 19.6,18.4 | 19.6,18.4 19.6,18.3 | 19.6,17.5 19.6,17.4 | 19.6,17.4 19.5,17.4 | 19.5,17.4 16.2,17.4 16,17.6 | 19.6,18.4 20.6,17.4 19.6,17.4 | 19.5,17.4 19.5,18 19.6,18.1 | 19.6,18.1 19.7,18.1 20.3,17.5 19.8,17.5 19.7,17.6 19.7,17.9 19.8,17.9 20,17.7 19.8,17.7
N$10
  Bottom 0.2: 20.1,4.1 19.1,4.1 19.1,5 | 19.1,5 18.8,5.3 | 19.1,5 19.8,4.3 19.4,4.3 19.2,4.5 19.2,4.6
N$11
  Bottom 0.2: 20.8,11.7 20.8,9 | 20.8,9 20.8,8.7 | 20.8,8.7 20.8,8.4 | 20.8,8.4 20.8,8.1 20.9,8.1 20.9,11 21.4,11.5 | IC4.6 17.7,11.77 17.7,12 | 17.7,12 17.5,12 | 17.5,12 17.5,11.5 19.5,11.5 | 19.5,11.5 19.8,11.5 | 19.8,11.5 19.8,11.6 20.2,11.6 | 20.6,11.6 20.7,11.6 | 20.7,11.6 21.3,11.6 | 21.3,11.6 21.3,11.8 | 21.3,11.8 21.3,12 | 21.3,12 21.5,13.1 | 21.5,13.1 23.84,13.1 IC4.2 | 17.8,11.9 17.6,11.9 17.5,12 | 17.7,12 20.9,12 | 20.9,12 21.2,12 | 21.2,12 21.3,12 | 21.3,12 21.2,11.9 19.6,11.9 19.6,11.6 19.5,11.5 | 19.8,11.5 20.6,11.5 | 20.6,11.5 21.1,11.5 | 21.1,11.5 21.3,11.5 | 21.3,11.5 21.3,11.6 | 21.3,11.8 21,11.8 | 19.5,11.8 21,11.8 | 21,11.8 21.3,11.5 | 21.4,11.5 21.4,12.8 | 21.4,12.8 21.4,12.9 | 21.4,12.9 21.4,13.1 21.5,13.1 | 21.5,13.1 21.2,12 | 21.5,13.1 21.8,13.3 | 21.8,13.3 25.1,13.3 | 25.1,13.3 25.1,12.7 | 25.1,12.7 21.5,12.7 21.4,12.8 | 21.4,12.8 21.8,12.8 | 21.8,12.8 24,12.8 | 24.2,12.8 24,12.8 | 24,12.8 23.8,13 21.5,13 21.4,12.9 | 21.8,13.3 21.5,13.3 21.2,13 21.2,12.3 20.9,12 | 20.6,11.5 20.7,11.6 | 20.7,11.6 20.7,8.7 | 20.7,8.7 20.7,8.6 | 20.7,8.6 20.7,7.6 20.28,7.6 R3.1 | 21.4,11.5 21.3,11.5 | 21.1,11.5 21.1,11.4 20.9,11.2 20.9,11.4 20.8,11.4 20.6,11.6 | 20.6,11.6 20.2,11.6 | 20.2,11.6 20.6,11.2 20.6,11.4 | 20.8,9 20.3,8.5 20.5,8.5 20.7,8.7 | 20.7,8.6 19.3,8.6 19.2,8.7 | 20.8,8.7 19.2,8.7 | 19.2,8.7 19.2,6.9 20.9,6.9 20.9,8.3 20.8,8.4 | 20.8,8.4 19.4,8.4 19.3,8.5 19.3,7 19.4,6.9 | 25.1,12.7 25.6,12.7 | 25.8,12.7 26.2,12.3 | 26.2,12.3 26.4,12.1 | 26.4,12.1 27.2,11.3 | 27.2,11.3 27.7,10.8 | 27.7,10.8 28.1,10.8 | 28.1,10.8 28.9,10.8 29.2,10.5 29.2,9.48 R4.2 | 25.1,13.3 25.2,13.3 | 25.2,13.3 25.8,12.7 | 25.8,12.7 25.6,12.7 | 25.6,12.7 25.2,13.1 25.2,12.9 25.3,12.8 25.4,12.8 25.8,12.4
  Bottom 0.2: 26,12.2 26.7,11.5 | 29.4,11.1 29.6,11.1 29.9,10.8 | 29.9,10.8 29.9,8.6 28.5,8.6 28.4,8.7 | 28.4,8.7 28.4,10.5 | 28.4,10.5 28.1,10.8 | 27.7,10.8 27.4,10.8 27.1,11.1 | 27.1,11.1 29.4,11.1 | 29.4,11.1 29.8,10.7 | 29.8,10.7 29.8,10.3 28.6,10.3 28.5,10.4 28.5,10.6 28.2,10.9 27.8,10.9 | 27.8,10.9 27.7,11 29.2,11 29.3,10.9 | 29.4,10.8 29.6,10.6 | 29.6,10.6 29.6,10.5 | 29.6,10.5 29.6,10.4 29.5,10.4 | 29.1,10.4 28.7,10.4 28.6,10.5 28.6,10.7 | 28.6,10.7 28.6,10.9 29.3,10.9 | 29.3,10.9 29.4,10.8 | 29.4,10.8 29.4,10.6 | 29.4,10.6 29.4,10.5 29.5,10.4 | 29.5,10.4 29.1,10.4 | 29.1,10.4 28.8,10.7 29.2,10.7 29.3,10.8 29.3,10.7 | 29.3,10.7 29.4,10.6 | 29.4,10.6 28.7,10.6 | 27.2,11.3 29.5,11.3 | 29.5,11.3 29.9,10.9 | 29.9,10.9 29.9,10.8 | 21.8,12.8 21.3,12.3 | 22.1,12.9 21.2,12 | 29.5,11.3 30.4,11.3 30.4,8.5 | 30.4,8.5 28.5,8.5 | 28.5,8.5 28.4,8.6 | 28.4,8.6 28.4,8.7 | 28.4,10.5 28.6,10.7 | 28.6,10.7 29.3,10.7 | 29.3,10.7 29.8,11.2 29.9,11.2 | 29.9,11.2 30.2,11.2 30.2,8.8 | 30.2,8.6 30.2,8.8 | 30.2,8.8 30.1,8.9 30.1,11 | 30.1,11 30,11.1 30,8.7 30.1,8.6 | 28.7,9.1 28.7,8.9 28.4,8.6 | 28.5,8.5 28.6,8.4 | 28.6,8.4 30.4,8.4 | 30.4,8.4 30.4,8.5 | 30.4,8.4 30.4,8.3 28.7,8.3 28.6,8.4 | 30.1,11.1 30.1,11 | 30.1,11 29.9,10.8 | 29.8,10.7 29.6,10.5 | 29.6,10.6 29.6,10.9 29.8,11.1 | 25.2,13.3 26.3,13.3 26.4,13.2 26.4,12.1 | 26.2,12.3 26.2,13.2 25.5,13.2 25.5,13.1 26,12.6 26,13.1 25.7,13.1 25.9,12.9 | 25.8,12.7 25.8,12.4 | 25.8,12.4 26,12.2 | 26,12.2 26,11.5 26.7,11.5 | 26.7,11.5 27.1,11.1 | 27.1,11.1 27.1,11.2 26.6,11.7 26.1,11.7 26.1,11.9 | 26.1,12 26.1,11.9 | 26.1,11.9 26.2,11.8 | 27.8,10.9 28.3,10.4 28.3,8.7 28.4,8.6 | 29.9,11.2 29.9,10.9 | 29.9,10.8 29.8,10.7
N$13
  Bottom 0.2: 8.2,5.7 8.2,5.6 7,4.4
N$14
  Bottom 0.2: IC2.3 10.9,5.8 | 10.9,5.8 10.9,5.5 11.4,5 | 12.2,2.37 JP7.5 12.4,2.44 12.4,4.3 10.9,5.8
N$15
  Bottom 0.2: 5.3,4 5.3,4.1 5.5,4.3 5.5,4.9
N$16
  Bottom 0.2: IC2.1 13.54,8.2 14.54,7 17,4.6 17.2,4.4 17.2,2.45 JP7.7
N$17
  Bottom 0.2: 4.6,2.35 JP7.2 4.7,2.35 4.7,4.2 7.09,6.59 IC2.6
N$18
  Bottom 0.2: 46.7,15.8 46.8,15.7
N$19
  Bottom 0.2: 18.8,5.2 18.8,5.1 18.9,5
N$20
  Bottom 0.2: 54.5,24.4 54.5,24.3 | 54.5,24.3 54.9,23.9 54.9,23.2 55,23.1 56.2,23.1 56.4,23.3 56.4,26.4 54.9,26.4 | 54.4,24.4 54.5,24.3 | 54.9,26.4 54.9,26.3 | 54.9,26.3 54.9,23.4 55.1,23.2 55.1,23.3 | 55.1,23.3 55.1,23.8 54.7,24.2 54.7,25 54.4,25.3 | 52.6,24.7 52.6,24.3 | 52.6,24.3 50.3,24.3 50.3,24.5 | 50.3,24.6 50.3,25.3 54.4,25.3 | 54.4,25.3 55.1,25.3 | 55.4,26.2 55.1,26.2 55.1,25.7 | 55.4,26.2 55.7,26.2 | 55.9,26.2 56,26.2 | 56,26.2 56.3,26.2 | 56.3,26.2 56.3,23.3 56.2,23.3 | 55.9,23.3 55.7,23.3 | 55.7,23.3 55.3,23.3 | 55.1,25.3 55.1,25.7 | 52.2,24.5 52.4,24.5 52.6,24.3 | 52.6,24.3 55.2,24.3 | 55.2,24.3 55.4,24.3 55.5,24.4 55.2,24.4 55.1,24.5 50.3,24.5 | 50.3,24.5 50.3,24.6 | 50.3,24.6 50.4,24.7 55.3,24.7 | JP16.7 55.6,24.68 55.5,24.1 54.95,24.55 55.34,24.55 55.4,24.6 | 55.4,24.6 55.6,24.8 51.93,24.8 IC1.9 | 55.3,24.7 55.4,24.6 | 55.3,24.7 55.1,24.9 50.4,24.9 50.4,25.1 55.5,25.1 | 55.1,25.3 55.5,25.3 56.2,26 56.2,23.3 | 56.2,23.3 55.9,23.3 | 55.9,23.3 55.9,26.1 56,26.2 | 56,26.2 56,23.5 56.1,23.4 55.8,23.4 55.7,23.3 | 55.7,23.3 55.7,26.1 | 55.7,26.1 55.7,26.2 | 55.7,26.2 55.9,26.2 | 55.9,26.2 56.1,26 55.3,26 55,26.3 55,25.9 | 55,25.8 55,23.4 55.1,23.3 | 55.1,23.3 55.3,23.3 | 55.3,23.3 55.3,25.9 | 55.3,25.9 55.3,26.3 55.4,26.2 | 55.4,26.2 55.4,25.9 | 55.4,24.2 55.4,23.5 55.5,23.4 55.6,23.5 55.6,26 55.7,26.1 | 55.7,26.1 55.6,26.1 55.4,25.9 | 55.4,25.9 55.4,24.2 | 55.4,24.2 55.1,23.9 55.1,24.2 55.2,24.3 | 54.3,25 54.3,25.2 55,25.9 | 55,25.9 55,25.8 | 55,25.8 55.1,25.7 | 55.1,25.7 55,25.7 54.7,25.4 | 55.3,25.9 54.9,26.3 | 54.9,26.4 54.9,26.6 56.4,26.6 56.4,26.3 56.3,26.2
N$21
  Bottom 0.2: 68.9,26.3 68.9,26.4 | 68.9,26.5 68.8,26.3 | JP16.2 68.28,25.58 68.8,26.1 | 68.8,26.1 69.1,26.4 68.9,26.4 | 68.9,26.4 68.9,26.5 | 68.9,26.5 68.6,26.6 | 72.4,26.4 72.3,26.6 72.3,22.6 | 72.3,22.6 72.3,22.3 71.8,21.8 | 71.1,21.3 70.1,21.3 | 70,21.3 68.2,21.3 64.2,17.3 50.3,17.3 50.3,16.8 64.2,16.8 68.4,21 | 68.5,21.1 68.4,21 | 68.4,21 71.3,21 | 71.3,21 71.9,21.5 72.5,22.1 | 72.5,22.1 72.5,22.2 | 67.9,26.2 68.1,26.2 68.9,26.4 | 68.3,26.3 68.5,26.1 | 68.5,26.1 68.5,26.3 68.8,26.6 | 68.8,26.6 68.8,26.5 | 68.8,26.3 68.9,26.4 | 69,26.7 69,25.7 68.2,24.9 68.3,24.9 68.3,26.3 | 68.3,26.3 68.8,26.5 | 72.5,26.8 72.5,26.7 | 72.5,26.7 72.5,22.2 | 71.2,21.3 71.5,21.6 | 71.5,21.6 71.7,21.6 | 71.7,21.6 71.9,21.8 | 72.4,22.3 72.2,22.3 | 72.2,22.3 71.5,21.6 | 72.2,22.3 72.4,22.5 72.4,22.3 | 72.4,22.3 71.9,21.8 | 71.9,21.8 71.8,21.8 | 71.8,21.8 71.1,21.3 | 71.1,21.3 70.4,21.2 69.8,21.2 69.9,21.1 70,21.1 70.8,21.2 70.3,21.1 70.1,21.3 | 70.1,21.3 70,21.3 | 70,21.3 69.9,21.2 68.3,21.2 68.2,21.1 | 68.2,21.1 68.3,21.1 | 68.2,21.1 68.1,21.1 66.9,19.9 66.9,19.8 67,19.8 68.2,21 68.1,21 64.3,17.2 | 64.3,17.2 64.3,17.1 64.4,17.1 | 64.4,17.1 67,19.7 | 64.4,17.1 64.3,17 50.6,17 50.5,16.9 50.5,17.1 64.2,17.1 64.3,17.2 | 64.3,17.2 51.95,17.2 IC1.15 | 72.3,22.6 70.8,21.1 71.2,21.1 71.7,21.6 | 71.7,21.6 71.9,21.6 72.5,22.2 | 72.5,22.1 72.5,22 71.5,21 71.3,21 | 71.3,21 71.3,21.3 71.4,21.4 71.3,21.4 71.1,21.2 | 68.8,26.1 68.8,26.3 | 68.8,26.3 68.8,26.5 | 68.8,26.5 69,26.7 | 69,26.7 68.9,26.4 | 72.2,26.8 72.3,26.8 | 72.5,26.7 72.3,26.8 | 72.3,26.8 72.2,26.7 | 72.1,26.7 69,26.7 | 69,26.7 68.6,26.6 | 72.2,26.8 72.4,26.5 72.4,26.4 | 72.2,26.8 72.1,26.7 | 72.1,26.7 72.2,26.7 | 72.2,26.7 72.5,26.7
  Bottom 0.2: 72.1,26.7 72.4,26.4 | 68.5,26.1 67.9,26.1 67.5,26.5 67.5,26.6 68.6,26.6 | 68.6,26.6 68.8,26.6 | 68.6,26.6 68.8,26.8 | 68.8,26.8 72.5,26.8 | 68.8,26.8 68.9,26.9 72.4,26.9 72.5,26.8
N$22
  Bottom 0.2: 49.5,12.6 49.5,11.2 49.6,11.1
N$23
  Bottom 0.2: IC1.10 50.52,23.38 50.5,23.4 | 50.5,23.4 50.3,23.6 | 52.8,23.6 53,23.6 | 53,23.6 53,23.1 | 53,23.1 53,23 | 53,23 50.3,23 50.3,23.6 | 50.3,23.6 52.8,23.6 | 52.8,23.6 52.9,23.5 52.9,23.2 52.8,23.1 50.6,23.1 50.5,23.2 | 50.5,23.3 50.5,23.4 | 50.5,23.4 50.6,23.4 50.7,23.5 50.8,23.5 50.9,23.4 50.9,23.2 50.6,23.2 50.5,23.3 | 50.5,23.3 50.5,23.2 | 50.5,23.2 50.4,23.1 52.9,23.1 53,23 | 53,23 53.7,23 | 53.7,23 53.8,22.9 | 53.8,22.6 53.9,22.5 | 53.9,22.5 54,22.5 | 54,22.5 54.2,22.5 | 54.4,22.5 57.2,22.5 57.4,22.7 57.4,23.98 JP16.6 | 53,23.6 54.1,23.6 54.2,23.5 54.2,22.7 54.4,22.5 | 54.4,22.5 54.2,22.5 | 54.2,22.5 54.1,22.6 54.1,23.3 54,23.4 52.8,23.4 52.7,23.3 53.4,23.3 | 53.4,23.3 54,23.3 54.1,23.4 53.3,23.4 53,23.1 | 53,23.1 53.4,23.1 | 53.4,23.1 53.8,23.1 | 53.8,23.1 54,23.1 54,22.9 | 54,22.8 54,22.9 | 54,22.9 53.8,23.1 | 53.8,23.1 53.8,23 | 53.8,23 53.8,22.9 | 53.8,22.9 54,22.7 | 54,22.7 54,22.8 | 54,22.8 53.8,23 | 53.8,23 53.5,23 | 53.5,23 53.4,23.1 | 53.5,23 54,22.5 | 54,22.5 54,22.7 | 53.7,23 53.4,23.3 | 53.4,23.3 53.4,23 53.8,22.6 | 53.9,22.5 54,22.4 | 54,22.4 57.4,22.4 57.6,22.6 57.6,22.7 | 57.6,23 57.6,22.7 | 57.6,22.7 57.4,22.5 57.4,22.8 57.7,23.1 57.7,22.6 | 53.8,22.9 53.8,22.6 | 54,22.4 54.1,22.3 57.4,22.3 | 57.4,22.3 57.7,22.6 | 57.7,22.6 58.3,23.2 58.2,23.2 57.8,22.8 | 57.4,22.3 58.3,22.3 | 58.3,22.3 59,23 58.8,23 | 58.5,23 58.3,23 57.7,22.4 58.1,22.4 58.2,22.5 | 58.2,22.5 58.3,22.5 58.8,23 | 58.8,23 58.5,23 | 58.5,23 58,22.5 58.2,22.5 | 58.2,22.5 58.6,22.9 | 58.3,22.3 58.5,22.3 59,22.8 59,23.2
N$24
  Bottom 0.2: IC1.11 52.7,22.11 53,22.4 53.1,22.4 53.8,21.7 59.2,21.7 60,22.5 60,23.1 60.8,23.9 60.8,24.7 JP16.5
N$25
  Bottom 0.2: X1.1 24.58,4.62 23.8,5.4 21.2,5.4 20.5,6.1 19,6.1 18.4,6.7 18.4,10 18.7,10.3 IC4.5 18.61,10.4 17.6,10.4 17.7,10.3
N$26
  Bottom 0.2: 50.7,17.2 50.5,17.2 50.4,17.1
N$27
  Bottom 0.406: IC4.1 27.42,14.3 IC6.18
N$28
  Bottom 0.2: IC6.7 35.04,21.66 35.1,21.6 | 35.1,21.6 35,21.6 | 35,21.6 34.7,21.6 34.7,24.3 | 34.7,24.3 35.1,24.3 | 35.1,24.3 35.3,24.3 35.3,21.6 35.2,21.6 35.2,24 | 35.2,24 35.2,24.1 34.9,24.1 | 34.9,24.1 34.9,21.7 | 34.9,24.1 34.9,24.2 35,24.2 35.2,24 | 35.2,24 35.1,24 35.1,21.7 35,21.6 | 35.1,21.6 35.4,21.6 35.4,25.7 37.9,25.7 38.7,24.9 | 39.4,24.2 39.5,24.1 39.5,20.3 39.6,20.2 | 39.4,24.2 39.4,20.2 39.6,20 42.3,20 43,19.3 47.2,19.3 47.2,19.8 43,19.8 42.5,20.3 39.8,20.3 39.7,20.4 39.7,24.2 | 39.7,24.2 39.7,24.3 | 39.7,24.3 38.9,25.1 | 34.7,25.1 34.7,24.9 | 34.7,24.3 34.7,24.7 | 34.7,24.7 34.7,24.9 | 34.7,24.9 34.8,25 | 35.3,24.6 34.9,24.6 34.8,24.7 34.9,24.8 | 34.9,24.8 34.8,24.9 34.8,24.4 35.3,24.4 35.3,24.8 | 35.3,24.8 35.3,24.9 | 35.3,24.9 35.1,24.9 | 35.1,24.9 34.9,24.9 34.7,25.1 | 39.7,24.3 39.7,24.4 38.2,25.9 34.7,25.9 | 39.7,24.2 39.6,24.2 38.8,25 | 38.8,25 38.8,24.8 | 38.8,24.8 39.4,24.2 | 39.6,20.2 39.7,20.3 39.6,20.3 39.6,20.2 | 39.6,20.2 42.3,20.2 43.1,19.4 44.7,19.4 44.7,19.6 43.1,19.6 42.5,20.2 42.5,19.9 42.7,19.7 45.49,19.7 IC1.4 | 35.1,24.3 34.7,24.7 | 34.7,25.1 34.7,25.9 | 34.8,25.8 34.7,25.9 | 38.7,24.9 38.8,24.8 | 38.7,24.9 38.8,24.9 38.9,25 38.8,25 | 38.8,25 38,25.8 | 38,25.8 38.1,25.8 38.8,25.1 | 38,25.8 35.8,25.8 | 35.8,25.8 34.9,25.8 34.9,24.8 | 34.9,24.8 35,24.7 35.2,24.7 35.3,24.8 | 35.3,24.9 35.3,25.6 35.2,25.7 35.1,25.7 35.1,24.9 | 35.2,25 35.2,25.2 35.8,25.8
N$29
  Bottom 0.2: IC1.12 51.34,20.84 51.1,20.6 52.7,20.6 | 52.7,20.6 52.7,20.5 | 52.7,20.5 52.6,20.5 | 52.6,20.5 50.3,20.5 50.3,21.1 52.9,21.1 53.2,20.8 61,20.8 62.6,22.4 62.6,23.4 62.7,23.5 62.7,23.2 62.9,23 62.9,22.3 61.2,20.6 60.9,20.6 | 60.9,20.6 52.7,20.6 | 52.7,20.6 52.6,20.5 | 52.7,20.5 61,20.5 | 61,20.5 61.1,20.5 | 61.1,20.5 63.8,23.2 63.8,24.1 JP16.4 | 60.9,20.6 61,20.5 | 61.1,20.5 61.6,20.5 | 61.6,20.5 61.7,20.5 | 61.7,20.5 64.2,23 63.8,23 61.5,20.7 61.5,20.6 | 61.5,20.6 61.6,20.6 63.9,22.9 | 61.5,20.6 61.6,20.5 | 61.7,20.5 61.8,20.5 64.2,22.9 64.2,23.3 64,23.5
N$30
  Bottom 0.2: 41.3,18.5 42.4,17.4
N$31
  Bottom 0.2: 29.3,11 29.6,10.7
N$32
  Bottom 0.2: 42.2,17.7 42.2,17.5 42.9,16.8 47.1,16.8 47.2,16.9 | IC6.9 37.58,23.22 37.5,23.3 | 37.3,23.5 38,23.5 | 38,23.5 38,22.3 | 37.3,23.5 37.3,21.6 | 37.3,21.6 37.5,21.6 | 37.5,21.6 38,21.6 | 38,21.6 38,22.3 | 38,22.3 37.9,22.4 37.5,22.4 37.4,22.3 37.4,21.7 37.8,21.7 37.9,21.8 37.9,22.2 37.7,22.2 | 37.7,22.2 37.5,22.2 37.5,21.8 | 37.5,21.8 37.7,21.8 | 37.7,21.8 37.8,21.9 37.8,22.1 37.7,22.2 | 37.7,22.2 37.7,22.1 37.6,22 37.6,21.9 | 38,21.6 38,19 38.4,18.6 41.4,18.6 42.98,17.02 | 42.98,17.02 43.2,16.8 47.2,16.8 47.2,16.9 | 47.2,16.9 47.2,17.1 | 47.2,17.1 47.2,17.3 42.4,17.3 41.3,18.4 38.3,18.4 37.8,18.9 37.8,21.8 37.7,21.8 | 37.5,21.8 37.3,21.6 | 37.3,21.6 37.3,21.5 37.9,20.9 37.9,21.2 37.5,21.6 | 37.5,21.6 37.4,21.5 37.5,21.4 | 37.5,21.4 37.7,21.2 | 47.2,16.9 42.9,16.9 42.6,17.2 43,17.2 | 43,17.2 47.1,17.2 47.2,17.1 | 47.2,17.1 43.1,17.1 43,17.2 | IC1.2 42.98,17.02 | 37.5,23.1 37.5,23.3 | 37.5,23.3 37.3,23.5 | 37.3,23.5 37.3,24.1 | 37.3,24.1 37.5,24.1 | 37.5,24.1 38,23.6 38,23.5 | 38,23.5 37.5,24 37.5,23.7 37.7,23.7 37.8,23.6 37.5,23.6 37.5,23.9 37.3,24.1 | 37.3,24.1 37.3,24.3 | 37.3,24.3 37.5,24.1 | 37.5,21.4 37.4,21.4 37.2,21.6 37.2,24.3 37.3,24.3
N$33
  Bottom 0.2: 25.8,12.6 27.5,10.9
N$34
  Bottom 0.2: 19.8,19.2 20.1,19.2 21.3,18 30.3,18 31,17.3 | 20.4,19 20.4,18.9 20.8,18.5 | 20.8,18.5 21.4,18.5 | 21.4,18.5 30.4,18.5 30.5,18.4 | 30.9,18 31,17.9 31,17.5 | 31,17.3 31,12.1 | 31,12.1 31.5,12.1 31.5,17.8 31.3,18 | 17.9,19.3 17.9,19.1 16.7,19.1 16.7,20 16.4,20.3 18.7,20.3 19.4,19.6 19.9,19.6 | 19.9,19.6 20.7,18.8 20.5,18.8 | Q1.3 19.9,19.4 20.2,19.1 | 20.5,18.8 20.6,18.7 20.8,18.7 | 20.8,18.7 21,18.7 | 21,18.7 30.6,18.7 31.3,18 | 31.3,18 31.3,13.38 IC6.15 | 20.5,18.8 20.2,19.1 | 20.2,19.1 17.4,19.1 17.2,19.3 17.2,19.6 16.7,20.1 18.8,20.1 19.1,19.8 16.9,19.8 | 16.8,19.8 16.9,19.8 | 16.9,19.8 17,19.9 18.8,19.9 | 31.3,18 31.1,18 30.5,18.6 30.5,18.5 31.1,17.9 31.1,17.7 | 31.1,17.7 31.1,17.1 | 31.1,17.1 31.1,12.2 31.4,12.2 31.4,12.4 | 31.4,13.1 31.4,12.4 | 31.4,12.4 31.3,12.3 31.3,13 | 31.3,13.1 31.3,13 | 31.3,13 31.2,12.9 | 31.2,12.9 31.2,14.7 | 31.2,12.9 31.2,12.3 31,12.1 | 31,12.1 30.9,12.1 30.9,18 | 19.9,19.6 20.4,19.6 | 20.4,19.3 20.4,19.1 20.8,18.7 | 20.8,18.7 20.8,18.8 20.3,19.3 20.3,19.4 20.2,19.5 20.3,19.5 20.4,19.4 | 20.4,19.4 20.4,19.6 | 20.4,19.4 20.4,19.3 | 20.4,19.3 21,18.7 | 21,18.7 20.8,18.5 | 20.8,18.5 20.9,18.4 21.1,18.4 | 21.1,18.4 30.4,18.4 | 30.4,18.4 30.5,18.4 | 30.5,18.4 30.9,18 | 30.4,18.4 31.1,17.7 | 31,17.3 31,17.5 | 31,17.5 30.3,18.2 21.2,18.2 21.1,18.3 | 21.1,18.4 21.1,18.2 21.6,17.7 30.5,17.7 31.1,17.1 | 21.4,18.5 21.4,18.6 20.4,19.6
N$35
  Bottom 0.2: R1.3 64.02,9.68 R2.2 63.08,9.7 57.5,9.7 IC5.4
N$37
  Bottom 0.2: 5.8,10.9 6.1,10.9 | 6.1,10.9 6.1,11 | 6.1,11 6.1,14 5.6,14 5.6,12.5 5.6,11.2 | 5.6,11.2 5.8,10.7 | 5.9,10.7 6.1,10.7 | 6.1,10.7 6.1,10.9 | 6.1,11 5.8,11 5.6,10.8 5.7,10.8 | 5.7,10.8 5.8,10.8 | 6.1,10.7 6.1,8.4 3,8.4 3,9.3 | 3,9.7 5.7,9.7 | 5.7,9.7 5.8,10.7 | 5.8,10.7 5.7,10.7 5.7,10 5.6,9.9 5.8,10.7 | 5.8,10.7 5.9,10.7 | 5.9,10.7 5.9,9.6 | 5.9,9.6 5.9,8.5 5.7,8.5 | 3.4,8.5 3.2,8.5 3.2,9.6 5.7,9.6 | 5.9,9.6 5.7,9.6 | 5.7,9.6 5.7,9.7 | 5.7,9.7 5.7,9.9 | 5.7,9.9 5.8,10.2 | 5.7,10.8 6,10.4 5.8,10.2 | 5.7,9.6 5.7,9.2 | 5.7,9.2 5.7,9.1 | 5.7,9.1 5.7,8.5 | 5.7,8.5 3.4,8.5 | 3.4,8.5 3.4,8.8 | 3.4,8.8 3.4,9.5 4.9,9.3 | 4.9,9.3 5.6,9.5 5.6,9.4 5.5,9.4 | 3.7,9.4 3.6,9.4 3.6,9.3 | 3.6,9.3 3.5,9.3 3.5,8.6 5.5,8.6 5.5,8.8 | 5.5,8.9 5.5,9.4 | 5.5,9.4 3.7,9.4 | 3.7,9.4 3.7,8.9 | 3.7,8.7 3.7,8.9 | 3.7,8.9 5.5,8.9 | 5.5,8.9 5.5,8.8 | 5.5,8.8 3.8,8.8 | 3.4,8.8 3.8,8.8 | 3.8,8.8 3.8,9.1 5.7,9.1 | 5.7,9.2 3.6,9.2 3.6,9.3 | 3.3,9.3 3,9.3 | 3,9.3 3,9.7 | 3,9.7 3,9.8 5.3,9.8 | 5.3,9.8 5.4,9.8 | 5.4,9.8 5.7,9.9 | 4.9,9.3 5.4,9.8 | 5.8,10.2 5.4,9.8 | 5.8,10.7 5.6,10.1 | 5.4,9.8 5.6,9.8 5.6,11.2 | 5.6,11.2 5.6,10.1 | 5.6,10.1 5.3,9.8
N$38
  Bottom 0.2: 5.6,11.9 5.6,13.8 6,13.8 5.9,13.7 5.9,11.7 5.7,11.9 5.7,12.2 5.8,12.3 5.8,13.7
N$39
  Bottom 0.2: 51.5,22.2 50.3,22.2 | 50.3,22.2 50.3,22.4 53.1,22.4 53.6,21.9 | 50.3,22.2 50.3,21.8 53.1,21.8 53.5,21.4 59.3,21.4 | 59.3,21.4 60.3,22.4 | 60.3,22.4 60.3,22.6 | 60.3,22.7 60.3,23.2 60.4,23.3 60.3,23.3 60.1,23.1 60.1,22.4 59.3,21.6 53.8,21.6 53.2,22.2 53,22.2 53,22.1 | 53,22.1 52.9,22 53.2,22 53.6,21.6 53.7,21.6 53.8,21.5 53.5,21.5 53.1,21.9 53.1,22 53,22.1 | 53,22.1 52.7,22.1 | 50.4,22.1 52.7,22.1 | 52.7,22.1 52.9,21.9 50.4,21.9 | 60.3,22.4 61,23.1 60.8,23.1 60.3,22.6 | 60.3,22.6 60.3,22.7 | 60.3,22.7 60.5,22.9 | 60,21.4 61.6,23 61.4,23 59.9,21.5 59.6,21.5 61,22.9 | 59.3,21.4 60,21.4 | 60,21.4 60.3,21.4 61.6,22.7 61.6,23.6 61.5,23.7
N$40
  Bottom 0.2: 65.4,23.3 65.3,23.3 | 65.3,23.3 65.2,23.3 65.3,23.2 | 65.3,23.3 65.4,23.2 65.3,23.2 | 65.3,23.2 65.3,22.2 | 65.3,22.2 65.1,22 | 65.1,22 63.2,20.1 | 63.2,20.1 62.4,19.3 | 62.4,19.3 62.3,19.6 | 62.3,19.6 62.4,19.7 62.6,19.7 62.4,19.5 62.3,19.6 | 62.3,19.6 50.4,19.6 50.4,19.4 62.2,19.4 | 62.2,19.4 62.3,19.4 62.4,19.3 | 65,22 65.1,22 | 65.3,22.2 66.4,23.3 66.2,23.3 65.4,22.5 65.4,22.7 | 65.4,22.7 65.4,22.9 65.5,23 65.7,23 65.4,22.7 | 65.1,23.7 65,23.6 65,22.3 62.5,19.8 | IC1.13 50.34,19.57 50.3,19.6 | 50.3,19.6 50.3,19.8 50.5,19.8 | 62.5,19.8 62.6,19.8 65.1,22.3 65.1,23.1 65,23.2 65.74,23.94 JP16.3 | 62.5,19.8 50.5,19.8 | 50.5,19.8 50.3,19.6 | 50.3,19.6 50.3,19.3 62.3,19.3 | 62.3,19.3 62.4,19.3 | 62.4,19.3 65.2,22.2 65.2,23.2 65.3,23.3 | 62.5,19.3 66.4,23.2 | 62.2,19.4 62.3,19.3 | 62.5,19.3 62.8,19.3 | 63.2,20.1 63.2,19.8 | 63.2,19.8 62.8,19.4 | 66.4,23.1 66.4,22.9 | 66.4,22.9 62.8,19.3 | 66.4,22.9 66.6,23.1 66.5,23.1 63.2,19.8 | 62.4,19.3 62.5,19.3 | 62.8,19.3 62.9,19.3 66.6,23 66.6,23.4 66.5,23.5
N$41
  Bottom 0.2: 4.6,13.7 4.6,12.5
N$42
  Bottom 0.2: 7,12.5 7,13.9 7.3,13.9 7.2,13.8 7.2,12.1
N$43
  Bottom 0.2: 7,11.5 6.8,11.3 6.8,7.1 | 6.8,7 6.8,6.7 4.4,4.3 4.5,4.3 6.9,6.7 7,6.7 | 7,6.7 7.1,6.6 4.5,4 4.5,4.2 7,6.7 | 7,6.7 7.1,6.7 7.2,6.8 | 7.2,6.8 7.2,6.7 | 7.2,6.8 7.2,7.6 | 7.2,7.6 7.2,10.9 7,10.9 7,7.1 | 7,7.1 7,6.7 | 4.2,4.1 4.2,4.3 7,7.1 | 7,7.1 6.8,7.1 | 6.8,7.1 6.7,7.1 | 6.7,7.1 3.9,4.3 | 6.7,7.1 7.2,7.6 | 4.8,4.1 4.8,5.1 6.8,7.1 | 6.8,7.1 6.8,7 | 6.8,7 4,4.2
N$44
  Bottom 0.2: 64,18.5 64,18.6 67.7,22.3
N$45
  Bottom 0.2: 10.8,12.3 10.8,13.8 10.9,13.8 11,13.9 10.8,13.9 10.7,13.8 11.1,13.8 11.1,12.3 10.9,12.1 10.9,13.6 11,13.7
N$46
  Bottom 0.2: 22.3,11.9 22.3,11.8 22.1,11.6
N$47
  Bottom 0.2: 7.8,4.1 8,4.1 8.1,4.2 8.1,4.5 | 8.1,4.8 8.1,4.5 | 8.1,4.5 8,4.4
N$48
  Bottom 0.2: 11.9,3.7 11.9,4.4 11.5,4.8 11.5,4.2 11.6,4.1 11.6,4.4 11.7,4.5 | 10.7,11.8 10.7,11.4 | 10.7,11.4 10.7,10.9 | 10.7,10.9 10.6,10.9 | 10.6,10.9 10.6,14 11.2,14 11.2,5.7 12.6,4.3 12.5,4.3 11.1,5.7 11.1,5.5 12.3,4.3 12.1,4.3 10.8,5.6 | 10.6,10.9 10.6,5.6 11.7,4.5 | 11.7,4.5 11.8,4.4 | 10.7,5.6 10.7,10.9 | 10.7,11.4 10.8,11.4 | 10.8,11.4 10.9,11.4 11,11.3 11,5.7 10.9,5.7 10.8,5.8 10.8,11.4
N$49
  Bottom 0.2: 12,10.8 12,7 12.4,6.6 12.4,10.5 | 12,12 12,12.3 11.9,12.4 11.9,14 12.5,14 12.5,10.6 | 12.5,10.6 12.4,10.5 | 12.4,10.5 11.9,10.5 | 11.9,10.5 11.9,13.7 12.1,13.9 12.1,10.7 12,10.6 | 12,10.6 12.2,10.6 | 12.2,10.6 12.3,10.7 | 12.3,13.9 12.3,10.7 | 12.3,10.7 12.4,10.6 12.3,10.6 | 12.3,10.6 12.2,10.6 | 12,10.6 11.9,10.5 | 11.9,10.5 11.9,6.8 14.4,4.3 | 12.5,10.6 12.5,6.9 15.1,4.3 14.9,4.3 12.5,6.7 12.5,6.5 12.4,6.4 12.5,6.4 14.6,4.3 | JP7.6 | IC2.2 12.38,6.6 13.07,6 14.6,4.4 14.6,4.3 | JP7.6 | 14.6,4.3 14.6,2.51 JP7.6 | 12.4,10.5 12.3,10.6 | 12.3,10.6 12.3,10.5 12.1,10.3 12.1,7 12.3,6.8 12.3,7.2 | 12.3,7.2 12.3,8.2 12.2,8.3 12.2,7.7 | 12.2,7.5 12.2,7.1 12,6.9 12,6.8 12.3,6.5 | 15.4,4.2 15.3,4.2 12.3,7.2 | 12.3,7.2 12.7,7.2 | 12.7,7.2 15.6,4.3 | 12.7,7.2 12.2,7.7 | 12.2,7.7 12.2,7.5 | 12.2,7.5 15.4,4.3
N$50
  Bottom 0.2: 14.2,4.1 14.1,4.1 14,4.2 14,4.4 | 14,4.8 14,4.4 | 14,4.4 14.1,4.3 14.1,4.4
N$51
  Bottom 0.2: 42.8,18.5 47.1,18.5 47.1,18.2 43.1,18.2 43.1,18.3 43,18.4 46.9,18.4 47,18.3
N$52
  Bottom 0.2: 16.7,3.9 16.7,4 16.5,4.2 16.5,4.9 | 13.4,12.2 13.2,12.4 13.2,14 13.8,14 13.8,10.5 | 13.8,10.5 13.6,10.5 | 13.6,10.5 13.5,10.5 | 13.5,10.5 13.2,10.5 | 13.2,10.5 13.2,13.7 13.4,13.9 13.6,13.9 13.7,13.8 13.7,10.7 13.6,10.6 | 13.6,10.6 13.4,10.6 13.3,10.7 13.3,13.6 13.4,13.7 13.5,13.7 13.5,10.7 13.6,10.6 | 13.6,10.6 13.6,13.7 13.5,13.8 13.5,10.8 13.2,10.5 | 13.2,10.5 13.2,8 16.9,4.3 | 13.8,10.5 13.8,8.1 17.6,4.3 17.4,4.3 13.6,8.1 13.5,8 13.6,8 17.9,3.7 17.7,3.7 16.8,4.6 | 16.8,4.6 16.5,4.9 | 16.5,4.9 16.4,5 | 16.4,5 13.5,7.9 13.5,10.4 13.6,10.5 | 13.6,10.5 13.6,8.3 13.7,8.2 13.6,8.2 13.4,8 13.4,10.4 13.5,10.5 | 16.8,4.6 16.8,4.5 16.7,4.4 | 16.4,5 16.4,4.2 16.6,4
N$53
  Bottom 0.2: 1.5,4 1.5,4.1 1.3,4.3 1.3,6.3 | 1.3,6.3 2.4,6.3 | 2.4,6.3 2.5,6.3 | 2.5,6.3 2.9,6.3 | 2.9,6.3 2.9,6.1 | 2.9,6.1 2.9,4.2 1.7,4.2 1.6,4.3 | 1.6,4.3 1.5,4.4 1.5,6.2 1.7,6.2 | 2.4,6.2 2.6,6.2 | 2.6,6.2 2.7,6.1 | 2.7,6.1 2.7,4.4 2.5,4.4 | 2.3,4.4 1.8,4.4 1.7,4.5 1.7,6.1 1.9,6.1 | 1.9,6.1 2.7,6.1 | 2.7,6.1 2.8,6.2 2.7,6.2 | 2.7,6.2 2.6,6.2 | 2.1,6.2 2,6.2 | 2,6.2 1.9,6.1 | 1.9,6.1 1.9,5.9 | 1.9,5.4 1.9,4.6 1.6,4.3 | 1.6,4.3 1.7,4.3 2,4.6 2,5.3 | 2,5.3 2,5.9 2.1,6 2.4,6 | 2.4,6 2.6,6 2.6,4.5 2.5,4.4 | 2.5,4.4 2.3,4.4 | 2.3,4.4 2.1,4.6 2.1,5.7 2.4,6 | 2.4,6 2.4,5.7 | 2.4,4.5 2.4,5.7 | 2.4,5.7 2.2,5.9 2.2,4.6 2.3,4.5 2.3,5.5 1.9,5.9 | 1.9,5.9 1.9,5.4 | 1.9,5.4 2,5.3 | 2.8,6.1 2.9,6.1 | 2.9,6.3 2.9,7.7 1.3,7.7 | 1.3,7.7 1.3,6.3 | 1.3,6.3 1.4,6.2 1.4,6.4 1.5,6.5 | 2.6,7.5 2.7,7.5 | 2.7,7.5 2.7,7.4 | 2.7,7.1 2.7,6.5 | 2.7,6.5 1.5,6.5 | 1.5,6.5 1.5,6.8 | 1.5,7.4 1.4,7.5 1.6,7.5 | 2.7,7.5 2.8,7.5 2.8,6.3 2.7,6.2 | 2.7,6.2 2.7,6.5 | 2.7,6.5 2.5,6.7 2.2,6.7 | 2,6.7 1.6,6.7 1.5,6.8 | 1.5,6.8 1.5,7.4 | 1.5,7.4 1.6,7.5 | 1.6,7.5 2.6,7.5 | 2.6,7.5 2.7,7.4 | 2.7,7.4 2.7,7.1 | 2.7,7.1 1.6,7.1 1.4,7.3 1.7,7.3 | 1.7,7.3 2.4,7.3 | 2.4,7.3 2.5,7.2 | 2.5,7.2 2.5,6.9 | 2.5,6.9 2.5,6.8 | 2.5,6.8 2.6,6.7 | 1.5,7.6 1.4,7.6 1.3,7.7 | 1.3,7.7 0.7,7.7 0.7,0.2 1.3,0.2 | 1.4,1.3 1.4,1 1.3,0.9 | 1.3,0.9 1.3,0.7 | 1.3,0.6 1.3,0.2 | 1.3,0.2 2.9,0.2 2.9,0.7 | 2.9,0.9 2.9,0.7 | 2.9,0.7 1.3,0.7 | 1.3,0.7 1.3,0.6 | 1.3,0.6 2.7,0.6 2.8,0.5 2.8,0.4 1.4,0.4 | 1.3,0.9 1.3,7.5 1.2,7.6 1.2,0.4 1.1,0.3 1,0.3 1,7.5 1.1,7.6 1,7.6 0.9,7.5 | 0.9,7.5 0.9,7.6 | 0.9,7.5 0.9,0.3 | 2.6,7.3 2.4,7.3 | 1.7,7.3 1.7,7 | 1.7,6.6 1.7,6.2 | 1.7,6.2 1.8,6.2 | 1.8,6.2 2,6.2 | 2.1,6.2 2.3,6.2 | 2.3,6.2 2.4,6.3 | 2.4,6.3 2.4,7.1 2.5,7.2 | 2.5,7.2 2,7.2 1.8,7 1.8,6.2
  Bottom 0.2: 2.3,6.2 2.4,6.2 | 2.4,6.2 2.5,6.3 | 2.5,6.3 2.5,6.8 | 2.5,6.8 2.3,7 1.7,7 | 1.7,7 1.7,6.6 | 1.7,6.6 2.2,6.6 2.5,6.9 | 2.5,6.9 2,6.9 2.2,6.7 | 2.2,6.7 2.2,6.3 2.1,6.2 | 2.1,6.2 2.1,6.7 1.9,6.9 1.9,6.8 2,6.7 | 2,6.7 2.2,6.7 | 2.2,6.7 2.3,6.6
N$54
  Bottom 0.2: 2.6,12.4 2.6,12.5 | 2.6,12.4 2.4,12.3 | 2.6,12.4 3.3,12.4 | 2.6,12.4 2.4,12.4 | 1.9,12.4 1.9,12.5 2.6,12.5 | 2.6,12.5 3.3,12.5 | 3.3,12.5 3.3,12.3 | 3.3,12.3 3.1,12.3 2.7,12.3 | 2.7,12.3 2.5,12.3 | 2.5,12.3 2.4,12.3 | 2.4,12.3 1.9,12.3 1.9,12.4 | 1.9,12.4 2.4,12.4 | 2.4,12.4 2.5,12.3 | 2.5,12.3 2.6,12.4 | 2.6,12.4 2.7,12.3 | 3.3,12.5 3.4,12.5 3.4,12.3 3.3,12.3
N$55
  Bottom 0.2: 1.6,14.1 1.6,26.7 | 1.6,26.7 1.6,27.3 1.7,27.4 | 1.6,26.7 2.3,27.4 2.1,27.4 1.7,27
N$57
  Bottom 0.2: 48.2,22.1 48.2,22.2 48.3,22.3 42.9,22.3 | 42.9,22.3 42.9,22.4 47.8,22.4 | 42.9,22.3 42.9,21.9 | 42.9,21.9 48.2,21.9 48.2,21.8 42.9,21.8 42.9,21.9 | 47.8,22.4 48.2,22.4 | 48.4,22.8 48.2,22.8 47.8,22.4
N$58
  Bottom 0.2: 30.4,17.8 21.8,17.8 21.5,18.1
N$59
  Bottom 0.2: 46.4,19.6 47.1,19.6 47.1,19.5 46.6,19.5 46.5,19.4
N$60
